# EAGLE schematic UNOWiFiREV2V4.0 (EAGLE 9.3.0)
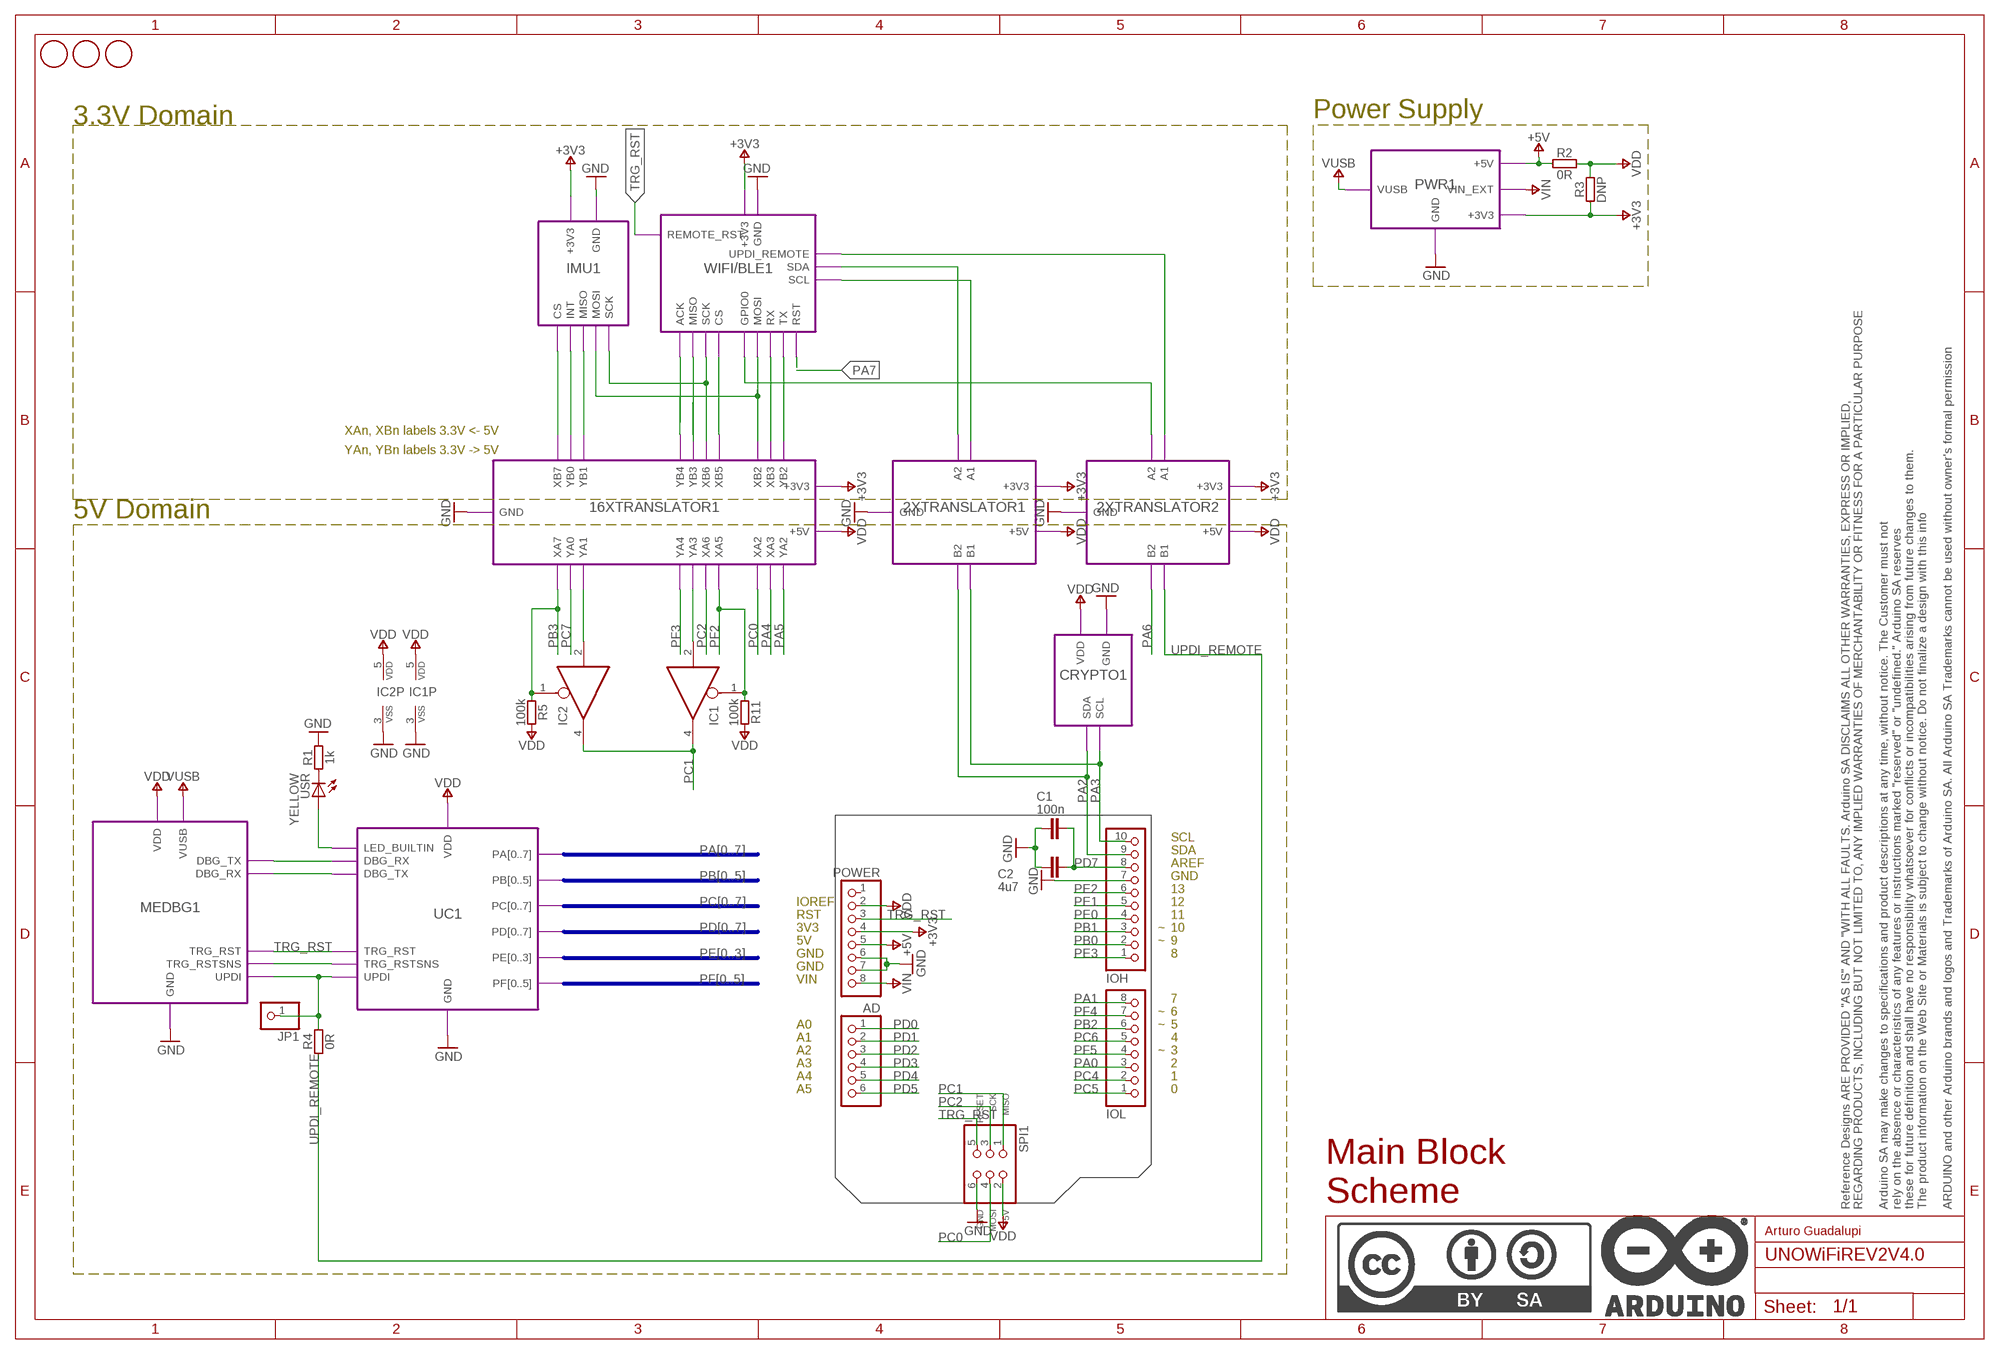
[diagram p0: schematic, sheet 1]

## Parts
AD  Analog  PINHD-1X06TH  [1X06-TH]
C1  100n  C-100NF-0402  [0402-1005X55N]
C2  4u7  C-4.7UF-0402  [0402-1005X55N]
FD1  DNP  FIDUCIAL-2MM  [FD-1-2]
FD2  DNP  FIDUCIAL-2MM  [FD-1-2]
FD3  DNP  FIDUCIAL-2MM  [FD-1-2]
FRAME1  DNP  A3-FRAME  [FRAME]
IC1  74LVC1G125DCKR  SN74LVC1G125DCKR  [SC70-5]
IC2  74LVC1G125DCKR  SN74LVC1G125DCKR  [SC70-5]
IOH  Digital  PINHD-1X10TH  [1X10]
IOL  Digital  PINHD-1X08-DIGITALTH  [1X08]
JP1  PINHD-1X1  [1X01]
POWER  Power  PINHD-1X08-POWERTH  [1X08]
R1  1k  R-1K-0402  [0402-1005X55N]
R2  0R  R-0R-0603  [C0603]
R3  DNP  RDNP-0603  [C0603]
R4  0R  R-0R-0402  [0402-1005X55N]
R5  100k  R-100K-0402  [0402-1005X55N]
R11  100k  R-100K-0402  [0402-1005X55N]
SPI1  -  PINHD-2X03-ICSPTH  [2X03]
USR  YELLOW  LED-YELLOW-0603  [LEDC1608X80N-AK]

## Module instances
UC1 = UC (part numbers offset by 900)
CRYPTO1 = CRYPTO (part numbers offset by 700)
MEDBG1 = MEDBG (part numbers offset by 800)
IMU1 = IMU (part numbers offset by 200)
2XTRANSLATOR1 = 2XTRANSLATOR (part numbers offset by 600)
WIFI/BLE1 = WIFI/BLE (part numbers offset by 300)
PWR1 = PWR (part numbers offset by 100)
16XTRANSLATOR1 = 16XTRANSLATOR (part numbers offset by 500)
2XTRANSLATOR2 = 2XTRANSLATOR (part numbers offset by 400)

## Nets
+3V3: POWER.4 R3.1 ; port WIFI/BLE1.+3V3 2XTRANSLATOR1.+3V3 PWR1.+3V3 IMU1.+3V3 16XTRANSLATOR1.+3V3 2XTRANSLATOR2.+3V3
+5V: POWER.5 R2.1 ; port PWR1.+5V
GND: C1.2 C2.2 IC1.3(VSS) IC2.3(VSS) IOH.7 POWER.6 POWER.7 R1.2 SPI1.6 ; port WIFI/BLE1.GND CRYPTO1.GND PWR1.GND MEDBG1.GND UC1.GND IMU1.GND 16XTRANSLATOR1.GND 2XTRANSLATOR1.GND 2XTRANSLATOR2.GND
N$1: port 2XTRANSLATOR2.A1 WIFI/BLE1.UPDI_REMOTE
N$2: port WIFI/BLE1.MISO 16XTRANSLATOR1.YB3
N$3: port WIFI/BLE1.TX 16XTRANSLATOR1.YB2
N$4: port IMU1.MOSI WIFI/BLE1.MOSI 16XTRANSLATOR1.XB2
N$5: port WIFI/BLE1.RX 16XTRANSLATOR1.XB3
N$6: port IMU1.MISO 16XTRANSLATOR1.YB1
N$7: port WIFI/BLE1.GPIO0 2XTRANSLATOR2.A2
N$8: port WIFI/BLE1.CS 16XTRANSLATOR1.XB5
N$9: IC1.2(I) ; port 16XTRANSLATOR1.YA3 16XTRANSLATOR1.YA3
N$10: IC2.2(I) ; port 16XTRANSLATOR1.YA1
N$12: port WIFI/BLE1.SCL 2XTRANSLATOR1.A1
N$13: port WIFI/BLE1.SDA 2XTRANSLATOR1.A2
N$14: JP1.1 R4.2 ; port UC1.UPDI MEDBG1.UPDI
N$15: port IMU1.INT 16XTRANSLATOR1.YB0
N$16: port IMU1.CS 16XTRANSLATOR1.XB7
N$17: port UC1.TRG_RSTSNS MEDBG1.TRG_RSTSNS
N$18: port WIFI/BLE1.ACK 16XTRANSLATOR1.YB4
N$19: port UC1.DBG_TX MEDBG1.DBG_RX
N$20: port MEDBG1.DBG_TX UC1.DBG_RX
N$21: USR.A ; port UC1.LED_BUILTIN
N$22: R1.1 USR.C
N$23: port IMU1.SCK WIFI/BLE1.SCK 16XTRANSLATOR1.XB6
PA0: IOL.3
PA1: IOL.8
PA2: IOH.9 ; port CRYPTO1.SDA 2XTRANSLATOR1.B2
PA3: IOH.10 ; port CRYPTO1.SCL 2XTRANSLATOR1.B1
PA4: port 16XTRANSLATOR1.XA3
PA5: port 16XTRANSLATOR1.YA2
PA6: port 2XTRANSLATOR2.B2
PA7: port WIFI/BLE1.RST
PB0: IOH.2
PB1: IOH.3
PB2: IOL.6
PB3: IC2.1(OE) R5.1 ; port 16XTRANSLATOR1.XA7
PC0: SPI1.4 ; port 16XTRANSLATOR1.XA2
PC1: IC1.4(O) IC2.4(O) SPI1.1
PC2: SPI1.3 ; port 16XTRANSLATOR1.XA6
PC4: IOL.2
PC5: IOL.1
PC6: IOL.5
PC7: port 16XTRANSLATOR1.YA0
PD0: AD.1
PD1: AD.2
PD2: AD.3
PD3: AD.4
PD4: AD.5
PD5: AD.6
PD7: C1.1 C2.1 IOH.8
PE0: IOH.4
PE1: IOH.5
PE2: IOH.6
PE3: IOH.1
PF2: IC1.1(OE) R11.1 ; port 16XTRANSLATOR1.XA5
PF3: port 16XTRANSLATOR1.YA4
PF4: IOL.7
PF5: IOL.4
TRG_RST: POWER.3 SPI1.5 ; port MEDBG1.TRG_RST UC1.TRG_RST WIFI/BLE1.REMOTE_RST
UPDI_REMOTE: R4.1 ; port 2XTRANSLATOR2.B1
VDD: IC1.5(VDD) IC2.5(VDD) POWER.2 R2.2 R3.2 R5.2 R11.2 SPI1.2 ; port CRYPTO1.VDD MEDBG1.VDD UC1.VDD 16XTRANSLATOR1.+5V 2XTRANSLATOR1.+5V 2XTRANSLATOR2.+5V
VIN: POWER.8 ; port PWR1.VIN_EXT
VUSB: port PWR1.VUSB MEDBG1.VUSB
Unconnected: POWER.1

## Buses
PA[0..7]
PB[0..5]
PC[0..7]
PD[0..7]
PE[0..3]
PF[0..5]

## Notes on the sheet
- 3.3V Domain | Power Supply
- XAn, XBn labels 3.3V <- 5V
- YAn, YBn labels 3.3V -> 5V
- 5V Domain
- SCL
- SDA
- AREF
- GND
- 13
- IOREF | 12
- RST | 11
- 3V3 | ~ | 10
- 5V | ~ | 9
- GND | 8
- GND
- VIN
- 7
- ~ | 6
- A0 | ~ | 5
- A1 | 4
- A2 | ~ | 3
- A3 | 2
- A4 | 1
- A5 | 0
- Main Block 
  Scheme
- Arturo Guadalupi

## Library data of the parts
AD = Arduino-connectors:PINHD-1X06: PIN HEADER; CODE-ARDUINO: 3649; DATASHEET: -; DISTRIBUTOR-LINK: -; DISTRIBUTOR-PN: -; MANUFACTURER: -; MANUFACTURER-PN: FH254-106DF085149V
C1 = Arduino-rcl:C: SMD Capacitor; CODE-ARDUINO: 0132; DATASHEET: http://www.tdk.com/pdf/TDKMLCCCapRange.pdf; DISTRIBUTOR-LINK: http://www.digikey.com/product-detail/en/tdk-corporation/C1005X5R1H104K050BB/445-5942-1-ND/2443982; DISTRIBUTOR-PN: 445-5942-1-ND; MANUFACTURER: TDK; MANUFACTURER-PN: C1005X5R1H104K050BB; NOTE: -
C2 = Arduino-rcl:C: SMD Capacitor; CODE-ARDUINO: 0833; DATASHEET: http://search.murata.co.jp/Ceramy/image/img/A01X/partnumbering_e_01.pdf; DISTRIBUTOR-LINK: http://www.digikey.com/product-detail/en/murata-electronics-north-america/GRM155R60J475ME47D/490-5915-1-ND/3719860; DISTRIBUTOR-PN: 490-5915-1-ND; MANUFACTURER: Murata; MANUFACTURER-PN: GRM155R60J475ME47D; NOTE: -
FD1-FD3 = Arduino-utility:FIDUCIAL: Fiducial mount; CODE-ARDUINO: DNP; DATASHEET: DNP; DISTRIBUTOR-LINK: DNP; DISTRIBUTOR-PN: DNP; MANUFACTURER: DNP; MANUFACTURER-PN: DNP
FRAME1 = Arduino-utility:A3-FRAME; CODE-ARDUINO: DNP; DATASHEET: DNP; DISTRIBUTOR-LINK: DNP; DISTRIBUTOR-PN: DNP; MANUFACTURER: DNP; MANUFACTURER-PN: DNP; NOTE: DNP
IC1 IC2 = Arduino-ICs:SN74LVC1G125DCKR: Single bus buffer with 3-state output; CODE-ARDUINO: 0040; DATASHEET: http://www.ti.com/lit/ds/symlink/sn74lvc1g125.pdf; DISTRIBUTOR-LINK: https://www.digikey.com/product-detail/en/texas-instruments/SN74LVC1G125DCKR/296-11604-1-ND/385743; DISTRIBUTOR-PN: 296-11604-1-ND; MANUFACTURER: Texas Instruments; MANUFACTURER-PN: SN74LVC1G125DCKR; NOTE: NO
IOH = Arduino-connectors:PINHD-1X10: PIN HEADER; CODE-ARDUINO: 3648; DATASHEET: -; DISTRIBUTOR-LINK: -; DISTRIBUTOR-PN: -; MANUFACTURER: -; MANUFACTURER-PN: FH254-110DF085149V
IOL = Arduino-connectors:PINHD-1X08: PIN HEADER; CODE-ARDUINO: 3648; DATASHEET: -; DISTRIBUTOR-LINK: -; DISTRIBUTOR-PN: -; MANUFACTURER: -; MANUFACTURER-PN: FH254-108DF085149V
JP1 = pinhead:PINHD-1X1: PIN HEADER
POWER = Arduino-connectors:PINHD-1X08: PIN HEADER; CODE-ARDUINO: 3649; DATASHEET: -; DISTRIBUTOR-LINK: -; DISTRIBUTOR-PN: -; MANUFACTURER: -; MANUFACTURER-PN: FH254-108DF085149V
R1 = Arduino-rcl:R: SMD Resistor; CODE-ARDUINO: 0140; DATASHEET: www.yageo.com.tw/exep/pages/download/literatures/PYu-R_INT-thick_7.pdf; DISTRIBUTOR-LINK: http://www.digikey.com/product-detail/en/yageo/RC0402FR-071KL/311-1.00KLRCT-ND/729460; DISTRIBUTOR-PN: 311-1.00KLRCT-ND; MANUFACTURER: Yageo; MANUFACTURER-PN: RC0402FR-071KL; NOTE: NO
R2 = Arduino-rcl:R: SMD Resistor; CODE-ARDUINO: 0233; DATASHEET: http://www.yageo.com/exep/pages/download/literatures/PYu-R_Marking_2.pdf; DISTRIBUTOR-LINK: https://www.digikey.com/product-detail/en/yageo/RC0603JR-070RL/311-0.0GRCT-ND/729622; DISTRIBUTOR-PN: 311-0.0GRCT-ND; MANUFACTURER: Yageo; MANUFACTURER-PN: RC0603JR-070RL; NOTE: NO
R3 = Arduino-rcl:R: SMD Resistor; CODE-ARDUINO: DNP; DATASHEET: DNP; DISTRIBUTOR-LINK: DNP; DISTRIBUTOR-PN: DNP; MANUFACTURER: DNP; MANUFACTURER-PN: DNP; NOTE: DNP
R4 = Arduino-rcl:R: SMD Resistor; CODE-ARDUINO: 0039; DATASHEET: www.yageo.com.tw/exep/pages/download/literatures/PYu-R_INT-thick_7.pdf; DISTRIBUTOR-LINK: http://www.digikey.com/product-detail/en/yageo/RC0402FR-070RL/311-0.0LRCT-ND/2827888; DISTRIBUTOR-PN: 311-0.0LRCT-ND; MANUFACTURER: Yageo; MANUFACTURER-PN: RC0402FR-070RL; NOTE: NO
R5 R11 = Arduino-rcl:R: SMD Resistor; CODE-ARDUINO: 0134; DATASHEET: www.yageo.com.tw/exep/pages/download/literatures/PYu-R_INT-thick_7.pdf; DISTRIBUTOR-LINK: http://www.digikey.com/product-detail/en/yageo/RC0402FR-07100KL/311-100KLRCT-ND/729473; DISTRIBUTOR-PN: 311-100KLRCT-ND; MANUFACTURER: Yageo; MANUFACTURER-PN: RC0402FR-07100KL; NOTE: NO
SPI1 = Arduino-connectors:PINHD-2X03-ICSP: PIN HEADER; CODE-ARDUINO: 0114; DATASHEET: -; DISTRIBUTOR-LINK: https://www.digikey.com/product-detail/en/samtec-inc/TSW-103-25-S-D/TSW-103-25-S-D-ND/7863771; DISTRIBUTOR-PN: TSW-103-25-S-D-ND; MANUFACTURER: Samtec; MANUFACTURER-PN: TSW-103-25-S-D
USR = Arduino-diodes:LED: LED; CODE-ARDUINO: 2243; DATASHEET: http://media.digikey.com/pdf/Data%20Sheets/Avago%20PDFs/HSMz-Czzz.pdf; DISTRIBUTOR-LINK: http://www.digikey.com/product-detail/en/broadcom-limited/HSMY-C190/516-1424-1-ND/637748; DISTRIBUTOR-PN: 516-1424-1-ND; MANUFACTURER: Avago; MANUFACTURER-PN: HSMY-C190

## Module UC
Ports: TRG_RSTSNS(out) UPDI(in) TRG_RST(in) GND(pwr) VDD(pwr) DBG_TX(out) DBG_RX(in) LED_BUILTIN(out) PC[0..7](io) PA[0..7](io) PB[0..5](io) PD[0..7](io) PE[0..3](io) PF[0..5](io)
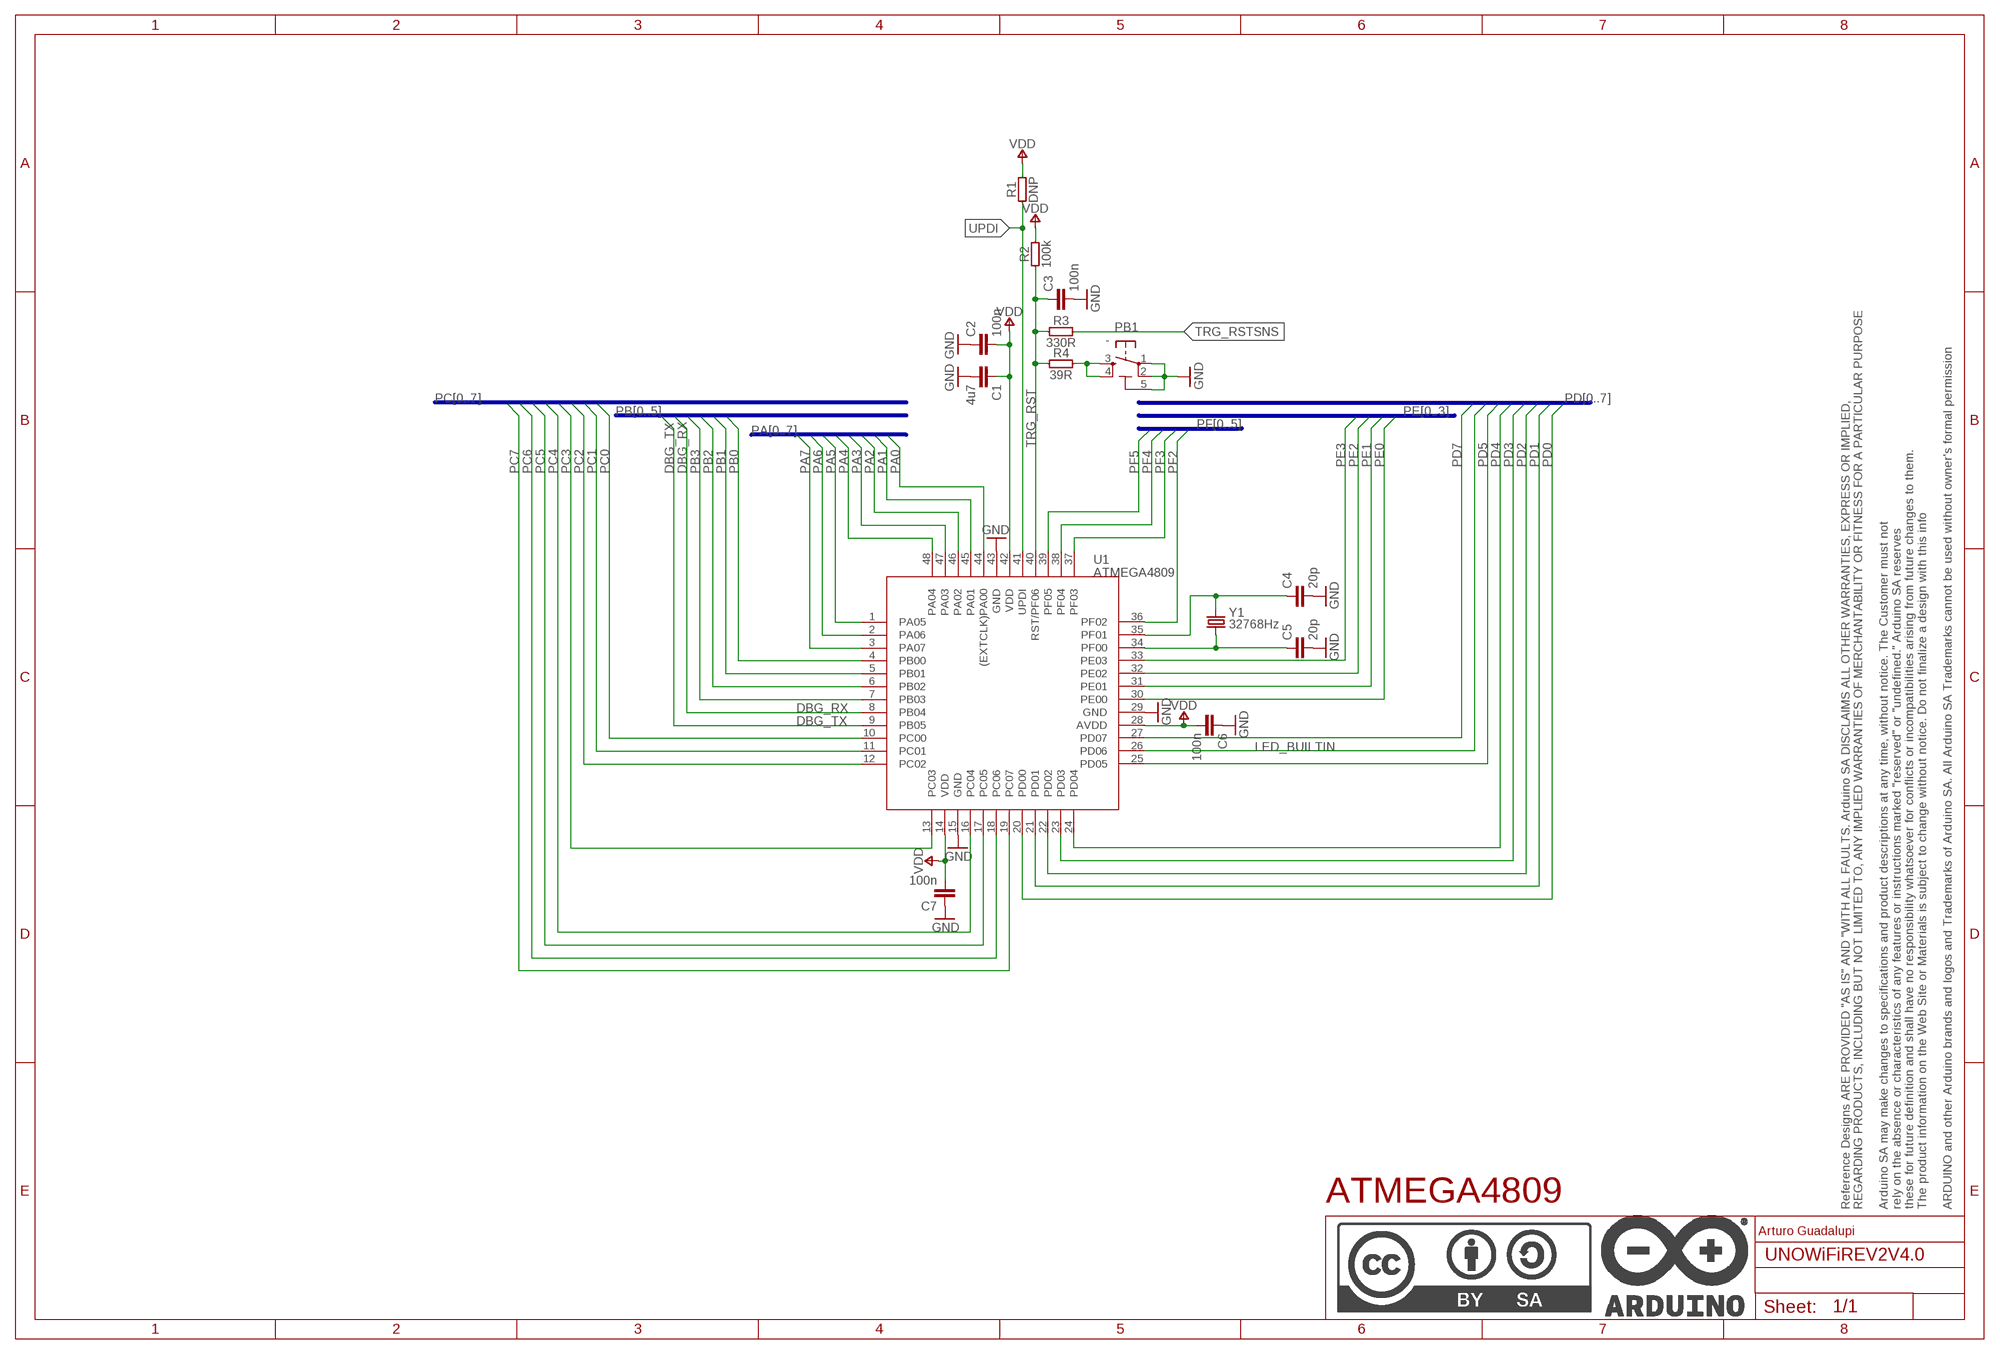
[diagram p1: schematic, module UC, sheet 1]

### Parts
C1  4u7  C-4.7UF-0402  [0402-1005X55N]
C2  100n  C-100NF-0402  [0402-1005X55N]
C3  100n  C-100NF-0402  [0402-1005X55N]
C4  20p  C-20PF-0402  [0402-1005X55N]
C5  20p  C-20PF-0402  [0402-1005X55N]
C6  100n  C-100NF-0402  [0402-1005X55N]
C7  100n  C-100NF-0402  [0402-1005X55N]
FRAME1  DNP  A3-FRAME  [FRAME]
PB1  -  TACTILE2  [TS42]
R1  DNP  R-DNP-0402  [0402-1005X55N]
R2  100k  R-100K-0402  [0402-1005X55N]
R3  330R  R-330R-0402  [0402-1005X55N]
R4  39R  R-39R-0402  [0402-1005X55N]
U1  ATMEGA4809  [TQFP48]
Y1  32768Hz  32.768KHZ  [ABS07]

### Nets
DBG_RX: U1.8(PB04)
DBG_TX: U1.9(PB05)
GND: C1.2 C2.1 C3.2 C4.2 C5.2 C6.1 C7.1 PB1.1 PB1.2 PB1.5(5-GND) U1.15(GND) U1.29(GND) U1.43(GND)
LED_BUILTIN: U1.26(PD06)
N$2: PB1.3 PB1.4 R4.2
N$3: C5.1 U1.34(PF00) Y1.1
N$4: C4.1 U1.35(PF01) Y1.2
PA0: U1.44((EXTCLK)PA00)
PA1: U1.45(PA01)
PA2: U1.46(PA02)
PA3: U1.47(PA03)
PA4: U1.48(PA04)
PA5: U1.1(PA05)
PA6: U1.2(PA06)
PA7: U1.3(PA07)
PB0: U1.4(PB00)
PB1: U1.5(PB01)
PB2: U1.6(PB02)
PB3: U1.7(PB03)
PC0: U1.10(PC00)
PC1: U1.11(PC01)
PC2: U1.12(PC02)
PC3: U1.13(PC03)
PC4: U1.16(PC04)
PC5: U1.17(PC05)
PC6: U1.18(PC06)
PC7: U1.19(PC07)
PD0: U1.20(PD00)
PD1: U1.21(PD01)
PD2: U1.22(PD02)
PD3: U1.23(PD03)
PD4: U1.24(PD04)
PD5: U1.25(PD05)
PD7: U1.27(PD07)
PE0: U1.30(PE00)
PE1: U1.31(PE01)
PE2: U1.32(PE02)
PE3: U1.33(PE03)
PF2: U1.36(PF02)
PF3: U1.37(PF03)
PF4: U1.38(PF04)
PF5: U1.39(PF05)
TRG_RST: C3.1 R2.1 R3.1 R4.1 U1.40(RST/PF06)
TRG_RSTSNS: R3.2
UPDI: R1.1 U1.41(UPDI)
VDD: C1.1 C2.2 C6.2 C7.2 R1.2 R2.2 U1.14(VDD) U1.28(AVDD) U1.42(VDD)

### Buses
PA[0..7]
PB[0..5]
PF[0..5]
PE[0..3]
PD[0..7]
PC[0..7]

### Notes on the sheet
- ATMEGA4809
- Arturo Guadalupi

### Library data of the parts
C1 = Arduino-rcl:C: SMD Capacitor; CODE-ARDUINO: 0833; DATASHEET: http://search.murata.co.jp/Ceramy/image/img/A01X/partnumbering_e_01.pdf; DISTRIBUTOR-LINK: http://www.digikey.com/product-detail/en/murata-electronics-north-america/GRM155R60J475ME47D/490-5915-1-ND/3719860; DISTRIBUTOR-PN: 490-5915-1-ND; MANUFACTURER: Murata; MANUFACTURER-PN: GRM155R60J475ME47D; NOTE: -
C2 C3 C6 C7 = Arduino-rcl:C: SMD Capacitor; CODE-ARDUINO: 0132; DATASHEET: http://www.tdk.com/pdf/TDKMLCCCapRange.pdf; DISTRIBUTOR-LINK: http://www.digikey.com/product-detail/en/tdk-corporation/C1005X5R1H104K050BB/445-5942-1-ND/2443982; DISTRIBUTOR-PN: 445-5942-1-ND; MANUFACTURER: TDK; MANUFACTURER-PN: C1005X5R1H104K050BB; NOTE: -
C4 C5 = Arduino-rcl:C: SMD Capacitor; CODE-ARDUINO: 2188; DATASHEET: http://www.kemet.com/docfinder?Partnumber=CBR04C200J5GAC; DISTRIBUTOR-LINK: http://www.digikey.com/product-detail/en/kemet/CBR04C200J5GAC/399-6173-1-ND/2732143; DISTRIBUTOR-PN: 399-6173-1-ND; MANUFACTURER: Kemet; MANUFACTURER-PN: CBR04C200J5GAC; NOTE: -
FRAME1 = Arduino-utility:A3-FRAME; CODE-ARDUINO: DNP; DATASHEET: DNP; DISTRIBUTOR-LINK: DNP; DISTRIBUTOR-PN: DNP; MANUFACTURER: DNP; MANUFACTURER-PN: DNP; NOTE: DNP
PB1 = Arduino-pushbuttons:TACTILE2: Pushbutton; CODE-ARDUINO: 0946; DATASHEET: http://www.mouser.com/ds/2/418/NG_CD_1571636_C1-122399.pdf; DISTRIBUTOR-LINK: https://www.mouser.it/ProductDetail/TE-Connectivity/1571636-3/?qs=%2fha2pyFaduiys%2fNUBzym%252bcoSb9tuK3Sjuv54qjf0hQ0%3d; DISTRIBUTOR-PN: 506-1571636-3; MANUFACTURER: TE; MANUFACTURER-PN: 1571636-3; PN-ALTERNATIVE1: TS42031-160WWS027260
R1 = Arduino-rcl:R: SMD Resistor; CODE-ARDUINO: DNP; DATASHEET: DNP; DISTRIBUTOR-LINK: DNP; DISTRIBUTOR-PN: DNP; MANUFACTURER: DNP; MANUFACTURER-PN: DNP; NOTE: NO
R2 = Arduino-rcl:R: SMD Resistor; CODE-ARDUINO: 0134; DATASHEET: www.yageo.com.tw/exep/pages/download/literatures/PYu-R_INT-thick_7.pdf; DISTRIBUTOR-LINK: http://www.digikey.com/product-detail/en/yageo/RC0402FR-07100KL/311-100KLRCT-ND/729473; DISTRIBUTOR-PN: 311-100KLRCT-ND; MANUFACTURER: Yageo; MANUFACTURER-PN: RC0402FR-07100KL; NOTE: NO
R3 = Arduino-rcl:R: SMD Resistor; CODE-ARDUINO: 2229; DATASHEET: www.yageo.com.tw/exep/pages/download/literatures/PYu-R_INT-thick_7.pdf; DISTRIBUTOR-LINK: http://www.digikey.com/product-detail/en/yageo/RC0402FR-07330RL/311-330LRCT-ND/729541; DISTRIBUTOR-PN: 311-330LRCT-ND; MANUFACTURER: Yageo; MANUFACTURER-PN: RC0402FR-07330RL; NOTE: NO
R4 = Arduino-rcl:R: SMD Resistor; CODE-ARDUINO: 0138; DATASHEET: www.yageo.com.tw/exep/pages/download/literatures/PYu-R_INT-thick_7.pdf; DISTRIBUTOR-LINK: http://www.digikey.com/product-detail/en/yageo/RC0402FR-0739RL/311-39.0LRCT-ND/729549; DISTRIBUTOR-PN: 311-39.0LRCT-ND; MANUFACTURER: Yageo; MANUFACTURER-PN: RC0402FR-0739RL; NOTE: NO
U1 = Arduino-ucs&SoCs:ATMEGA4809: ATMEGA4809; CODE-ARDUINO: 2322; DATASHEET: http://ww1.microchip.com/downloads/en/DeviceDoc/40002016A.pdf; DISTRIBUTOR-LINK: https://www.digikey.com/product-detail/en/microchip-technology/ATMEGA4809-AFR/ATMEGA4809-AFRCT-ND/8540756; DISTRIBUTOR-PN: ATMEGA4809-AFRCT-ND; MANUFACTURER: Microchip; MANUFACTURER-PN: ATMEGA4809-AFR
Y1 = Arduino-crystals:32.768KHZ: LF crystal; CODE-ARDUINO: 0213; DATASHEET: http://www.abracon.com/Resonators/ABS07.pdf; DISTRIBUTOR-LINK: http://www.digikey.com/product-detail/en/abracon-llc/ABS07-32.768KHZ-T/535-9542-1-ND/1237009; DISTRIBUTOR-PN: 535-9542-1-ND; MANUFACTURER: Abracon LLC; MANUFACTURER-PN: ABS07-32.768KHZ-T

## Module CRYPTO
Ports: SDA(io) SCL(in) GND(pwr) VDD(pwr)
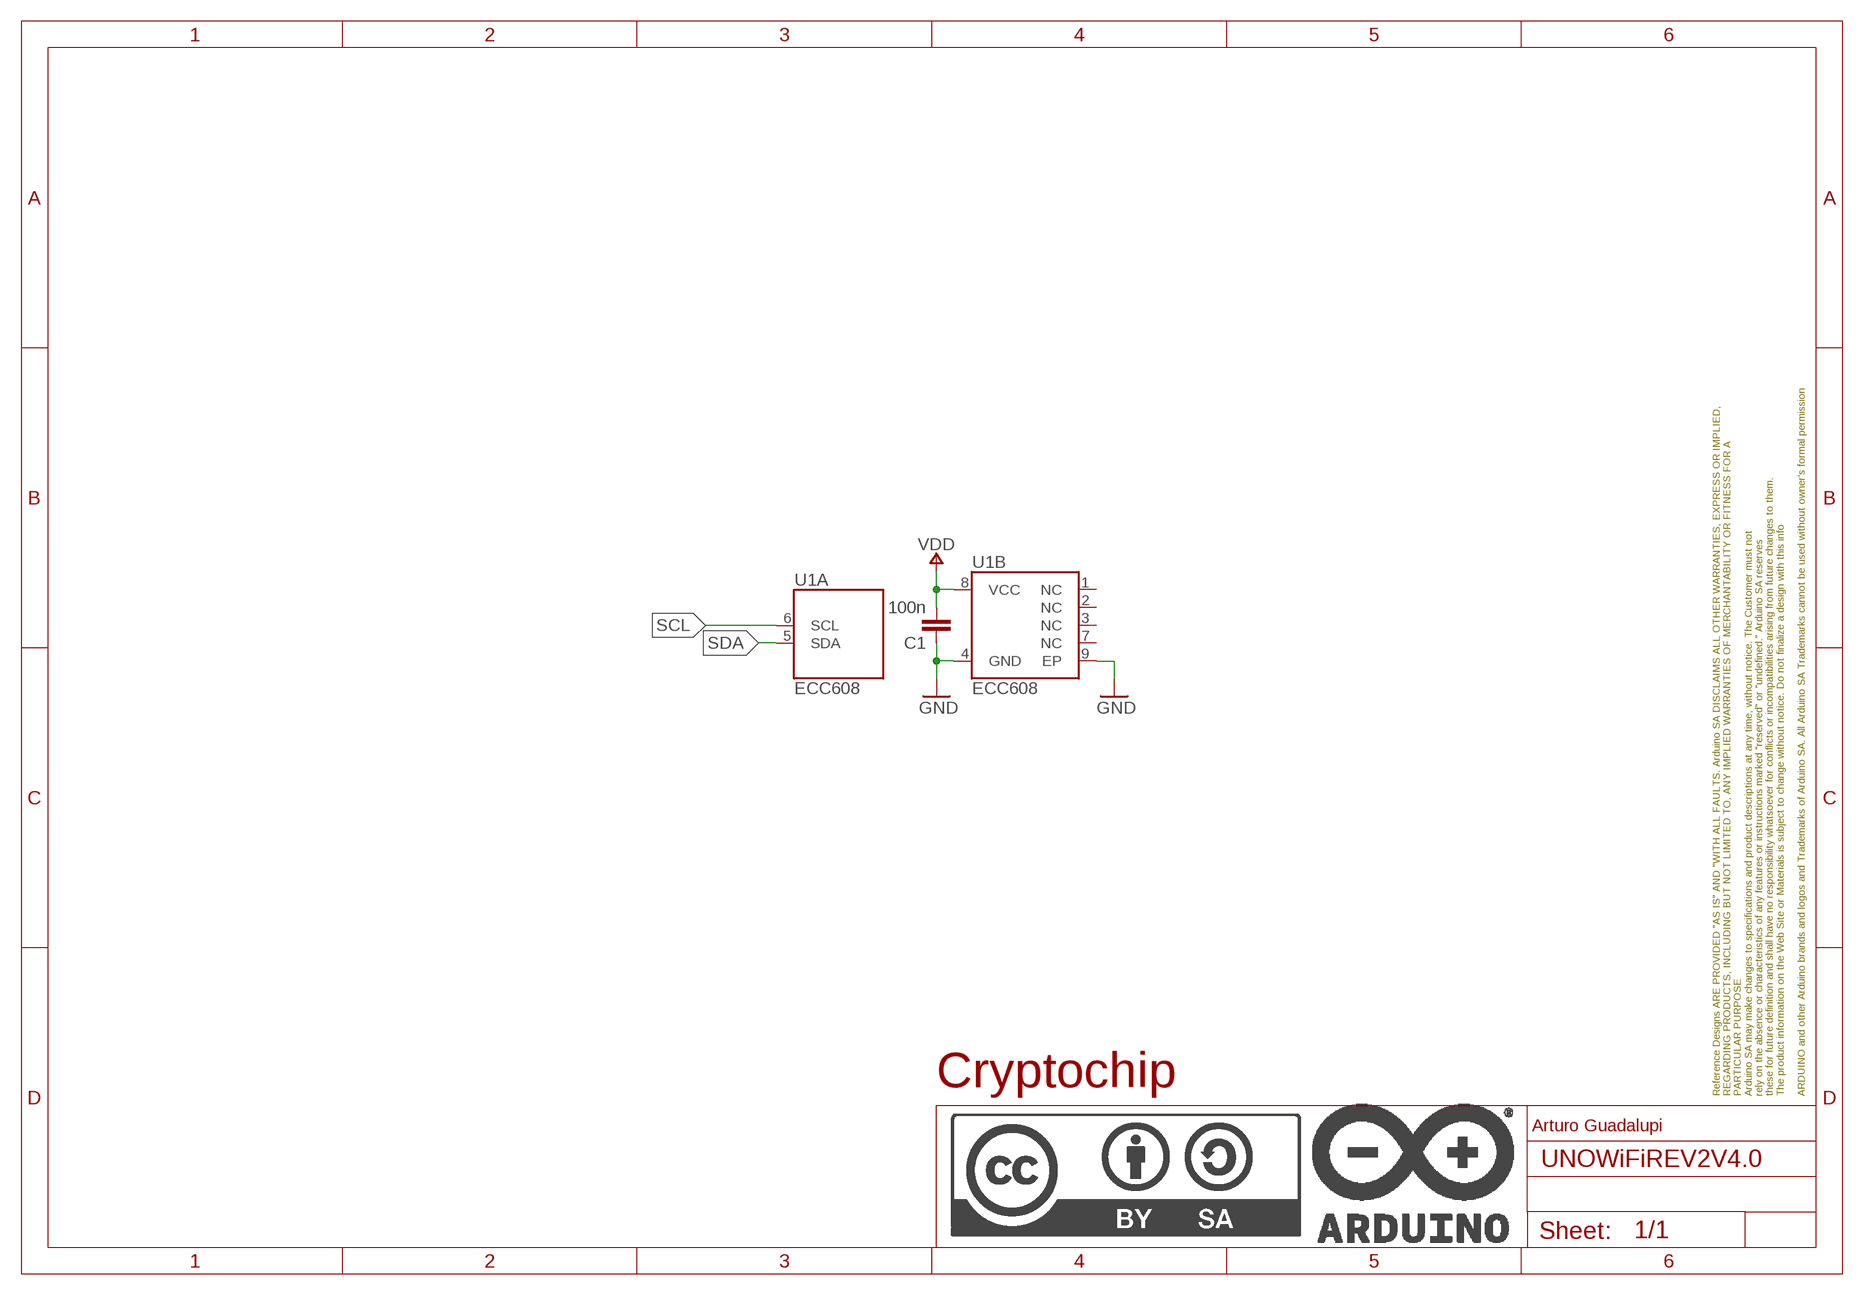
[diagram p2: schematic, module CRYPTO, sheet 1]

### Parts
C1  100n  C-100NF-0402  [0402-1005X55N]
FRAME1  DNP  A4L-LOC  [FRAME]
U1  ECC608  ATECC-6088-UDFN  [SON50P300X200X60-9N-EP160X140]

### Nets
GND: C1.1 U1.4(B:GND) U1.9(B:EP)
SCL: U1.6(A:SCL)
SDA: U1.5(A:SDA)
VDD: C1.2 U1.8(B:VCC)
Unconnected: U1.1(B:NC) U1.2(B:NC) U1.3(B:NC) U1.7(B:NC)

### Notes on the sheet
- Cryptochip
- Arturo Guadalupi

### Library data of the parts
C1 = Arduino-rcl:C: SMD Capacitor; CODE-ARDUINO: 0132; DATASHEET: http://www.tdk.com/pdf/TDKMLCCCapRange.pdf; DISTRIBUTOR-LINK: http://www.digikey.com/product-detail/en/tdk-corporation/C1005X5R1H104K050BB/445-5942-1-ND/2443982; DISTRIBUTOR-PN: 445-5942-1-ND; MANUFACTURER: TDK; MANUFACTURER-PN: C1005X5R1H104K050BB; NOTE: -
FRAME1 = Arduino-utility:A4L-LOC; CODE-ARDUINO: DNP; DATASHEET: DNP; DISTRIBUTOR-LINK: DNP; DISTRIBUTOR-PN: DNP; MANUFACTURER: DNP; MANUFACTURER-PN: DNP; NOTE: DNP
U1 = Arduino-ICs:ATECC: Secure authentication and product validation device, EEPROM, I2C, 2.0 - 5.5V; CODE-ARDUINO: A5007; DATASHEET: http://ww1.microchip.com/downloads/en/DeviceDoc/40001977A.pdf; DISTRIBUTOR-LINK: https://www.digikey.com/product-detail/en/microchip-technology/ATECC608A-MAHDA-T/ATECC608A-MAHDA-TCT-ND/7928236; DISTRIBUTOR-PN: ATECC608A-MAHDA-TCT-ND; MANUFACTURER: Microchip; MANUFACTURER-PN: ATECC608A-MAHDA-T; NOTE: NO

## Module MEDBG
Ports: VDD(pwr) VUSB(pwr) GND(pwr) DBG_TX(out) DBG_RX(in) TRG_RSTSNS(in) TRG_RST(out) UPDI(out)
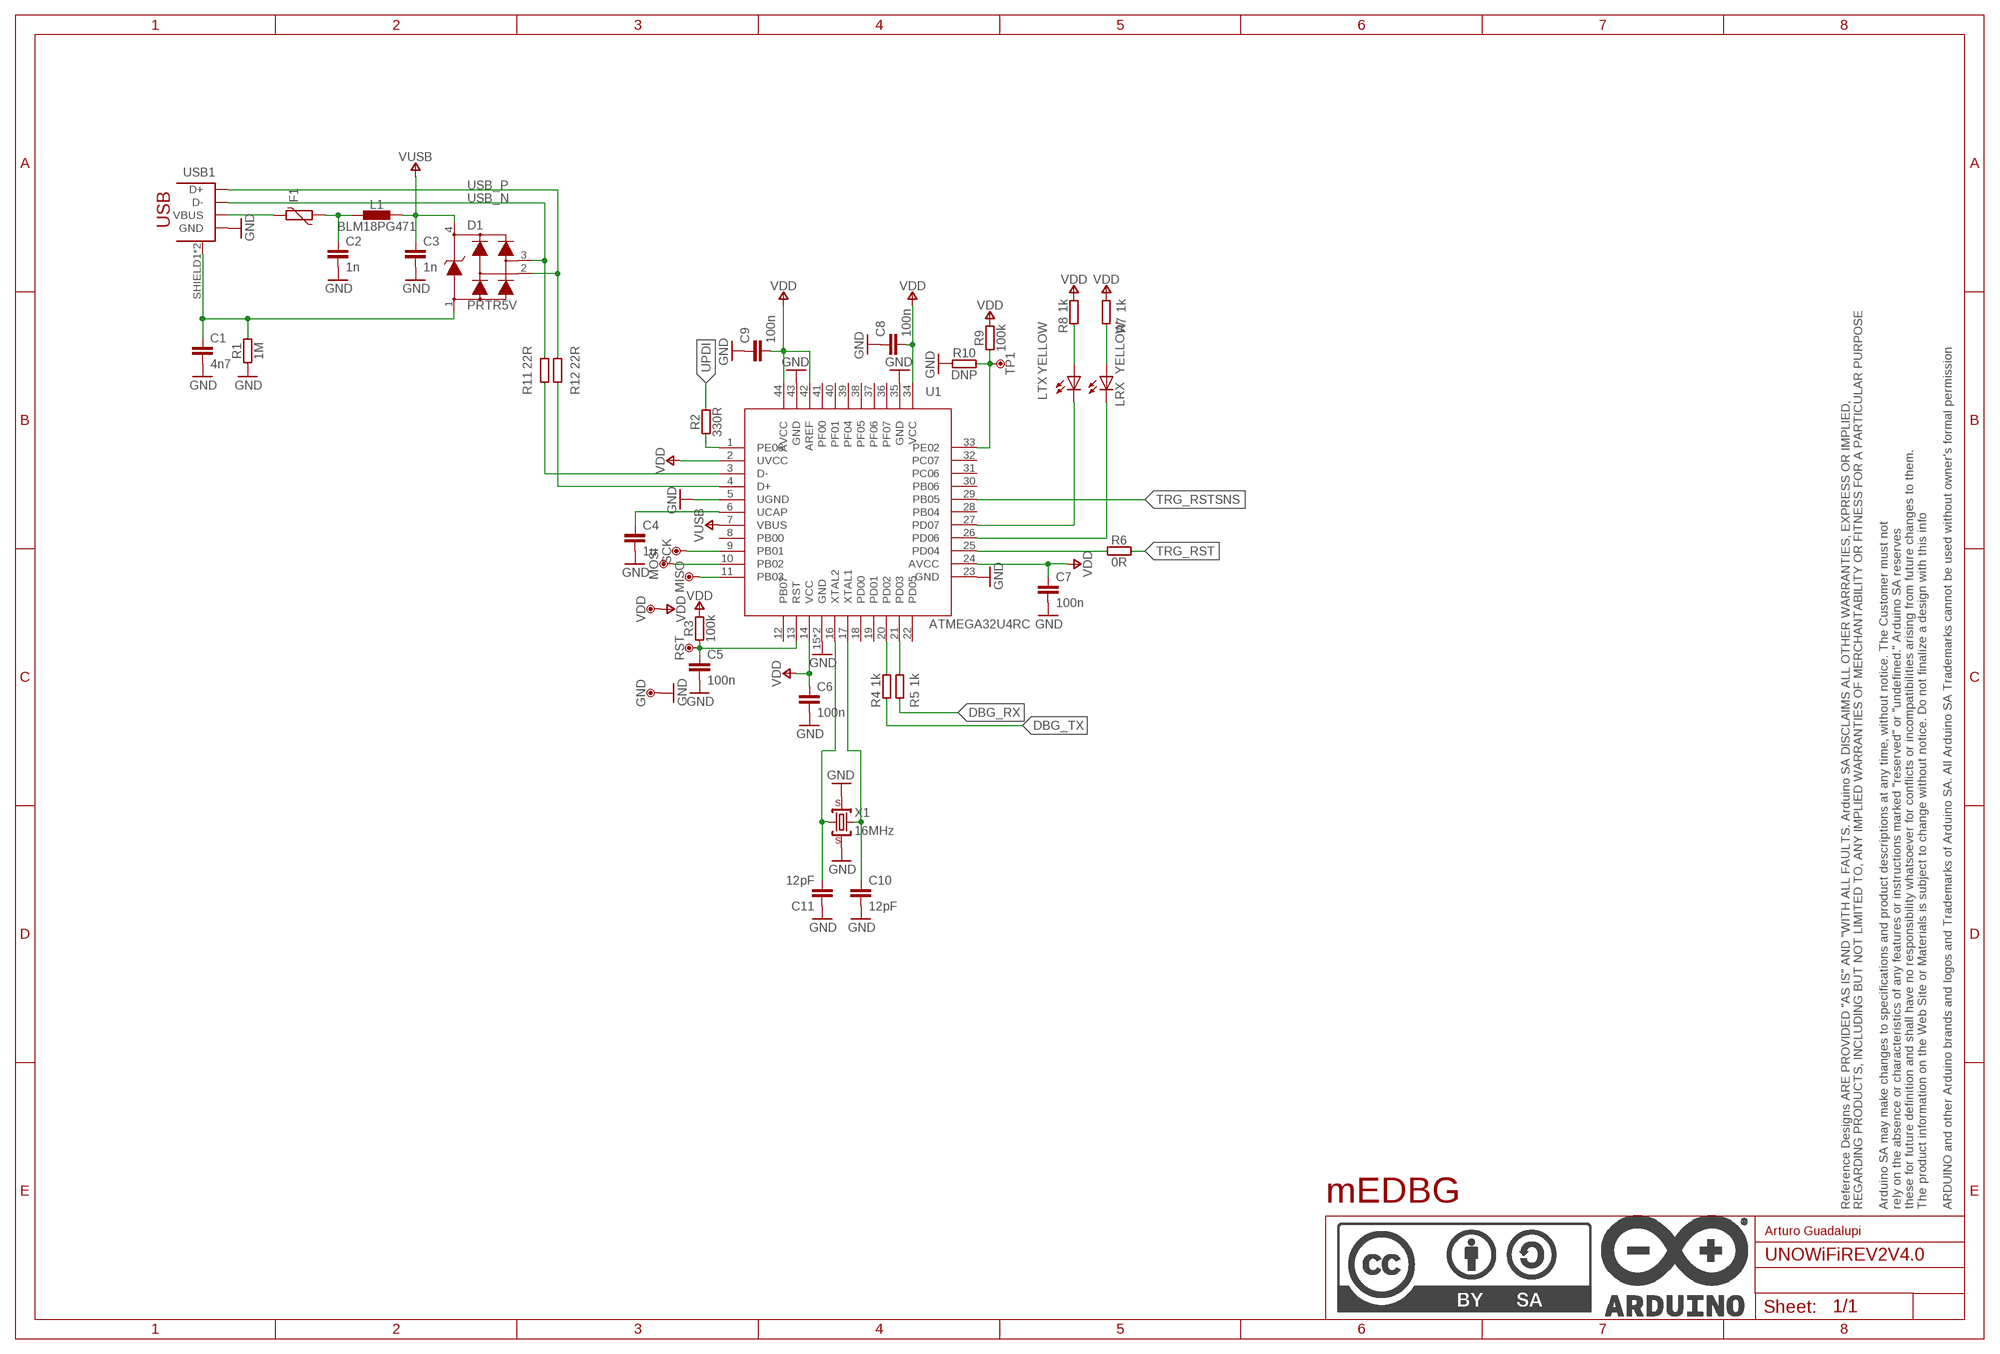
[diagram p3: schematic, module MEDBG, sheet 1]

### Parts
C1  4n7  C4.7NF-0805  [0805-R2013X50N]
C2  1n  C-1NF-0402  [0402-1005X55N]
C3  1n  C-1NF-0402  [0402-1005X55N]
C4  1u  C-1UF-0402  [0402-1005X55N]
C5  100n  C-100NF-0402  [0402-1005X55N]
C6  100n  C-100NF-0402  [0402-1005X55N]
C7  100n  C-100NF-0402  [0402-1005X55N]
C8  100n  C-100NF-0402  [0402-1005X55N]
C9  100n  C-100NF-0402  [0402-1005X55N]
C10  12pF  C-12PF-0402  [0402-1005X55N]
C11  12pF  C-12PF-0402  [0402-1005X55N]
D1  PRTR5V  PRTR5V0U2X,215  [SOT190P230X110-4N]
F1  PTC-0805  [C0805]
FRAME1  DNP  A3-FRAME  [FRAME]
GND  DNP  TPTP-1.00MM  [TP-1.00MM]
L1  BLM18PG471  FERRITE-470R0603  [0603-1608X90N]
LRX  YELLOW  LED-YELLOW-0603  [LEDC1608X80N-AK]
LTX  YELLOW  LED-YELLOW-0603  [LEDC1608X80N-AK]
MISO  DNP  TPTP-1.00MM  [TP-1.00MM]
MOSI  DNP  TPTP-1.00MM  [TP-1.00MM]
R1  1M  R-1M-0402  [0402-1005X55N]
R2  330R  R-330R-0402  [0402-1005X55N]
R3  100k  R-100K-0402  [0402-1005X55N]
R4  1k  R-1K-0402  [0402-1005X55N]
R5  1k  R-1K-0402  [0402-1005X55N]
R6  0R  R-0R-0402  [0402-1005X55N]
R7  1k  R-1K-0402  [0402-1005X55N]
R8  1k  R-1K-0402  [0402-1005X55N]
R9  100k  R-100K-0402  [0402-1005X55N]
R10  DNP  R-DNP-0402  [0402-1005X55N]
R11  22R  R-22R-0402  [0402-1005X55N]
R12  22R  R-22R-0402  [0402-1005X55N]
RST  DNP  TPTP-1.00MM  [TP-1.00MM]
SCK  DNP  TPTP-1.00MM  [TP-1.00MM]
TP1  DNP  TPTP-1.27MM  [TP-1.27MM]
U1  ATMEGA32U4RC  ATMEGA32U4  [QFN50P700X700X100-45N]
USB1  -  USB-B-H  [USB-B-H]
VDD  DNP  TPTP-1.00MM  [TP-1.00MM]
X1  16MHz  CRYSTAL-3.2X2.5-16MHZ(12PF)  [CRYSTAL-3.2-2.5]

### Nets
DBG_RX: R5.1
DBG_TX: R4.1
GND: C1.2 C2.2 C3.2 C4.2 C5.2 C6.2 C7.2 C8.1 C9.1 C10.2 C11.1 GND.X R1.1 R10.1 U1.5(UGND) U1.15(GND) U1.23(GND) U1.35(GND) U1.43(GND) U1.45(GND) USB1.GND X1.2(GND) X1.4(GND)
N$1: C1.1 D1.1 R1.2 USB1.SHIELD1(SHIELD) USB1.SHIELD2(SHIELD)
N$2: F1.2 USB1.VBUS
N$3: C2.1 F1.1 L1.1
N$4: R2.1 U1.1(PE06)
N$5: C4.1 U1.6(UCAP)
N$6: C5.1 R3.1 RST.X U1.13(RST)
N$7: C11.2 U1.16(XTAL2) X1.1(C1)
N$8: C10.1 U1.17(XTAL1) X1.3(C2)
N$9: R4.2 U1.20(PD02)
N$10: R5.2 U1.21(PD03)
N$11: LTX.C U1.27(PD07)
N$12: R6.1 U1.25(PD04)
N$13: LRX.C U1.26(PD06)
N$14: LTX.A R8.1
N$15: LRX.A R7.1
N$16: R9.1 R10.2 TP1.X U1.33(PE02)
N$17: MISO.X U1.11(PB03)
N$18: MOSI.X U1.10(PB02)
N$19: SCK.X U1.9(PB01)
TRG_RST: R6.2
TRG_RSTSNS: U1.29(PB05)
UPDI: R2.2
USB2_N: R11.1 U1.3(D-)
USB2_PI: R12.1 U1.4(D+)
USB_N: D1.3 R11.2 USB1.D-
USB_P: D1.2 R12.2 USB1.D+
VDD: C6.1 C7.1 C8.2 C9.2 R3.2 R7.2 R8.2 R9.2 U1.2(UVCC) U1.14(VCC) U1.24(AVCC) U1.34(VCC) U1.42(AREF) U1.44(AVCC) VDD.X
VUSB: C3.1 D1.4 L1.2 U1.7(VBUS)
Unconnected: U1.8(PB00) U1.12(PB07) U1.18(PD00) U1.19(PD01) U1.22(PD05) U1.28(PB04) U1.30(PB06) U1.31(PC06) U1.32(PC07) U1.36(PF07) U1.37(PF06) U1.38(PF05) U1.39(PF04) U1.40(PF01) U1.41(PF00)

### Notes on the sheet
- mEDBG
- Arturo Guadalupi

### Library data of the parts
C1 = Arduino-rcl:C: SMD Capacitor; CODE-ARDUINO: 0689; DATASHEET: http://www.kemet.com/Lists/ProductCatalog/Attachments/40/KEM_C1010_X7R_HV_SMD.pdf; DISTRIBUTOR-LINK: www.kemet.com/docfinder?Partnumber=C0805C472KDRACTU; DISTRIBUTOR-PN: 399-6738-1-ND; MANUFACTURER: Kemet; MANUFACTURER-PN: C0805C472KDRACTU; NOTE: -
C2 C3 = Arduino-rcl:C: SMD Capacitor; CODE-ARDUINO: 2321; DATASHEET: http://www.samsungsem.com/kr/support/product-search/mlcc/__icsFiles/afieldfile/2016/08/18/S_CL05B102KB5NNNC.pdf; DISTRIBUTOR-LINK: http://www.digikey.com/product-detail/en/samsung-electro-mechanics-america-inc/CL05B102KB5NNNC/1276-1032-1-ND/3889118; DISTRIBUTOR-PN: 1276-1032-1-ND; MANUFACTURER: Samsung; MANUFACTURER-PN: CL05B102KB5NNNC; NOTE: -
C4 = Arduino-rcl:C: SMD Capacitor; CODE-ARDUINO: 0133; DATASHEET: http://search.murata.co.jp/Ceramy/image/img/A01X/partnumbering_e_01.pdf; DISTRIBUTOR-LINK: http://www.digikey.com/product-detail/en/murata-electronics-north-america/GRM155R61E105KA12D/490-10017-1-ND/5026367; DISTRIBUTOR-PN: 490-10017-1-ND; MANUFACTURER: Murata; MANUFACTURER-PN: GRM155R61E105KA12D; NOTE: -
C5-C9 = Arduino-rcl:C: SMD Capacitor; CODE-ARDUINO: 0132; DATASHEET: http://www.tdk.com/pdf/TDKMLCCCapRange.pdf; DISTRIBUTOR-LINK: http://www.digikey.com/product-detail/en/tdk-corporation/C1005X5R1H104K050BB/445-5942-1-ND/2443982; DISTRIBUTOR-PN: 445-5942-1-ND; MANUFACTURER: TDK; MANUFACTURER-PN: C1005X5R1H104K050BB; NOTE: -
C10 C11 = Arduino-rcl:C: SMD Capacitor; CODE-ARDUINO: A5006; DATASHEET: http://search.murata.co.jp/Ceramy/image/img/A01X/partnumbering_e_01.pdf; DISTRIBUTOR-LINK: https://www.digikey.com/product-detail/en/murata-electronics-north-america/GJM1555C1H120GB01D/490-8078-1-ND/4380364; DISTRIBUTOR-PN: 490-8078-1-ND; MANUFACTURER: Murata; MANUFACTURER-PN: GJM1555C1H120GB01D; NOTE: -
D1 = Arduino-diodes:PRTR5V0U2X,215: USB ESD protection; CODE-ARDUINO: 2209; DATASHEET: http://www.nxp.com/documents/data_sheet/PRTR5V0U2X.pdf; DISTRIBUTOR-LINK: http://www.digikey.com/product-detail/en/nxp-semiconductors/PRTR5V0U2X,215/568-4140-1-ND/1589981; DISTRIBUTOR-PN: 568-4140-1-ND; MANUFACTURER: NXP; MANUFACTURER-PN: PRTR5V0U2X,215
F1 = Arduino-rcl:PTC: SMD PTC; CODE-ARDUINO: 0002; DATASHEET: https://www.bourns.com/docs/Product-Datasheets/mfmsmf.pdf; DISTRIBUTOR-LINK: https://www.digikey.it/product-detail/en/bourns-inc/MF-MSMF050-2/MF-MSMF050-2CT-ND/662842; DISTRIBUTOR-PN: MF-MSMF050-2CT-ND; MANUFACTURER: Bourns; MANUFACTURER-PN: MF-MSMF050-2
FRAME1 = Arduino-utility:A3-FRAME; CODE-ARDUINO: DNP; DATASHEET: DNP; DISTRIBUTOR-LINK: DNP; DISTRIBUTOR-PN: DNP; MANUFACTURER: DNP; MANUFACTURER-PN: DNP; NOTE: DNP
GND MISO MOSI RST SCK TP1 VDD = Arduino-utility:TP: Testpoint; CODE-ARDUINO: DNP; DATASHEET: DNP; DISTRIBUTOR-LINK: DNP; DISTRIBUTOR-PN: DNP; MANUFACTURER: DNP; MANUFACTURER-PN: DNP
L1 = Arduino-rcl:FERRITE: SMD ferrite; CODE-ARDUINO: 2217; DATASHEET: http://search.murata.co.jp/Ceramy/image/img/PDF/ENG/L0110S0100BLM18P.pdf; DISTRIBUTOR-LINK: http://www.digikey.com/product-detail/en/murata-electronics-north-america/BLM18PG471SN1D/490-5223-1-ND/1948399; DISTRIBUTOR-PN: 490-5223-1-ND; MANUFACTURER: Murata; MANUFACTURER-PN: BLM18PG471SN1D; NOTE: -
LRX LTX = Arduino-diodes:LED: LED; CODE-ARDUINO: 2243; DATASHEET: http://media.digikey.com/pdf/Data%20Sheets/Avago%20PDFs/HSMz-Czzz.pdf; DISTRIBUTOR-LINK: http://www.digikey.com/product-detail/en/broadcom-limited/HSMY-C190/516-1424-1-ND/637748; DISTRIBUTOR-PN: 516-1424-1-ND; MANUFACTURER: Avago; MANUFACTURER-PN: HSMY-C190
R1 = Arduino-rcl:R: SMD Resistor; CODE-ARDUINO: 0139; DATASHEET: www.yageo.com.tw/exep/pages/download/literatures/PYu-R_INT-thick_7.pdf; DISTRIBUTOR-LINK: http://www.digikey.com/product-detail/en/yageo/RC0402JR-07330RL/311-330JRCT-ND/729412; DISTRIBUTOR-PN: 311-330JRCT-ND; MANUFACTURER: Yageo; MANUFACTURER-PN: RC0402JR-07330RL; NOTE: NO
R2 = Arduino-rcl:R: SMD Resistor; CODE-ARDUINO: 2229; DATASHEET: www.yageo.com.tw/exep/pages/download/literatures/PYu-R_INT-thick_7.pdf; DISTRIBUTOR-LINK: http://www.digikey.com/product-detail/en/yageo/RC0402FR-07330RL/311-330LRCT-ND/729541; DISTRIBUTOR-PN: 311-330LRCT-ND; MANUFACTURER: Yageo; MANUFACTURER-PN: RC0402FR-07330RL; NOTE: NO
R3 R9 = Arduino-rcl:R: SMD Resistor; CODE-ARDUINO: 0134; DATASHEET: www.yageo.com.tw/exep/pages/download/literatures/PYu-R_INT-thick_7.pdf; DISTRIBUTOR-LINK: http://www.digikey.com/product-detail/en/yageo/RC0402FR-07100KL/311-100KLRCT-ND/729473; DISTRIBUTOR-PN: 311-100KLRCT-ND; MANUFACTURER: Yageo; MANUFACTURER-PN: RC0402FR-07100KL; NOTE: NO
R4 R5 R7 R8 = Arduino-rcl:R: SMD Resistor; CODE-ARDUINO: 0140; DATASHEET: www.yageo.com.tw/exep/pages/download/literatures/PYu-R_INT-thick_7.pdf; DISTRIBUTOR-LINK: http://www.digikey.com/product-detail/en/yageo/RC0402FR-071KL/311-1.00KLRCT-ND/729460; DISTRIBUTOR-PN: 311-1.00KLRCT-ND; MANUFACTURER: Yageo; MANUFACTURER-PN: RC0402FR-071KL; NOTE: NO
R6 = Arduino-rcl:R: SMD Resistor; CODE-ARDUINO: 0039; DATASHEET: www.yageo.com.tw/exep/pages/download/literatures/PYu-R_INT-thick_7.pdf; DISTRIBUTOR-LINK: http://www.digikey.com/product-detail/en/yageo/RC0402FR-070RL/311-0.0LRCT-ND/2827888; DISTRIBUTOR-PN: 311-0.0LRCT-ND; MANUFACTURER: Yageo; MANUFACTURER-PN: RC0402FR-070RL; NOTE: NO
R10 = Arduino-rcl:R: SMD Resistor; CODE-ARDUINO: DNP; DATASHEET: DNP; DISTRIBUTOR-LINK: DNP; DISTRIBUTOR-PN: DNP; MANUFACTURER: DNP; MANUFACTURER-PN: DNP; NOTE: NO
R11 R12 = Arduino-rcl:R: SMD Resistor; CODE-ARDUINO: 0468; DATASHEET: www.yageo.com.tw/exep/pages/download/literatures/PYu-R_INT-thick_7.pdf; DISTRIBUTOR-LINK: http://www.digikey.com/products/en?keywords=311-22.0LRCT-ND; DISTRIBUTOR-PN: 311-22.0LRCT-ND; MANUFACTURER: Yageo; MANUFACTURER-PN: RC0402FR-0722RL; NOTE: NO
U1 = Arduino-ucs&SoCs:ATMEGA32U4: ATMEGA32U4; CODE-ARDUINO: 0159; DATASHEET: http://ww1.microchip.com/downloads/en/DeviceDoc/Atmel-7766-8-bit-AVR-ATmega16U4-32U4_Datasheet.pdf; DISTRIBUTOR-LINK: https://www.digikey.com/product-detail/en/microchip-technology/ATMEGA32U4RC-MU/ATMEGA32U4RC-MU-ND/2507984; DISTRIBUTOR-PN: ATMEGA32U4RC-MU-ND; MANUFACTURER: Microchip; MANUFACTURER-PN: ATMEGA32U4RC-MU
USB1 = Arduino-connectors:USB: USB Connectors; CODE-ARDUINO: 0056; DATASHEET: http://cnctech.us/pdfs/1001-003-02000.pdf; DISTRIBUTOR-LINK: https://www.digikey.com/products/it?keywords=1001-003-02000; DISTRIBUTOR-PN: 1175-1002-ND; MANUFACTURER: CNC Tech; MANUFACTURER-PN: 1001-003-02000; PN-ALTERNATIVE1: USB-B-S-RA-WT-SPCC
X1 = Arduino-crystals:CRYSTAL-3.2X2.5: Crystal SMD 3.2x2.5mm; CODE-ARDUINO: 0395; DATASHEET: https://www.ecsxtal.com/store/pdf/ECX-33Q.pdf; DISTRIBUTOR-LINK: https://www.digikey.com/product-detail/en/ecs-inc/ECS-160-12-33Q-JES-TR/XC2147CT-ND/6050976; DISTRIBUTOR-PN: XC2147CT-ND; MANUFACTURER: ECS; MANUFACTURER-PN: ECS-160-12-33Q-JES-TR

## Module IMU
Ports: MOSI(in) SCK(in) MISO(out) INT(out) CS(in) +3V3(pwr) GND(pwr)
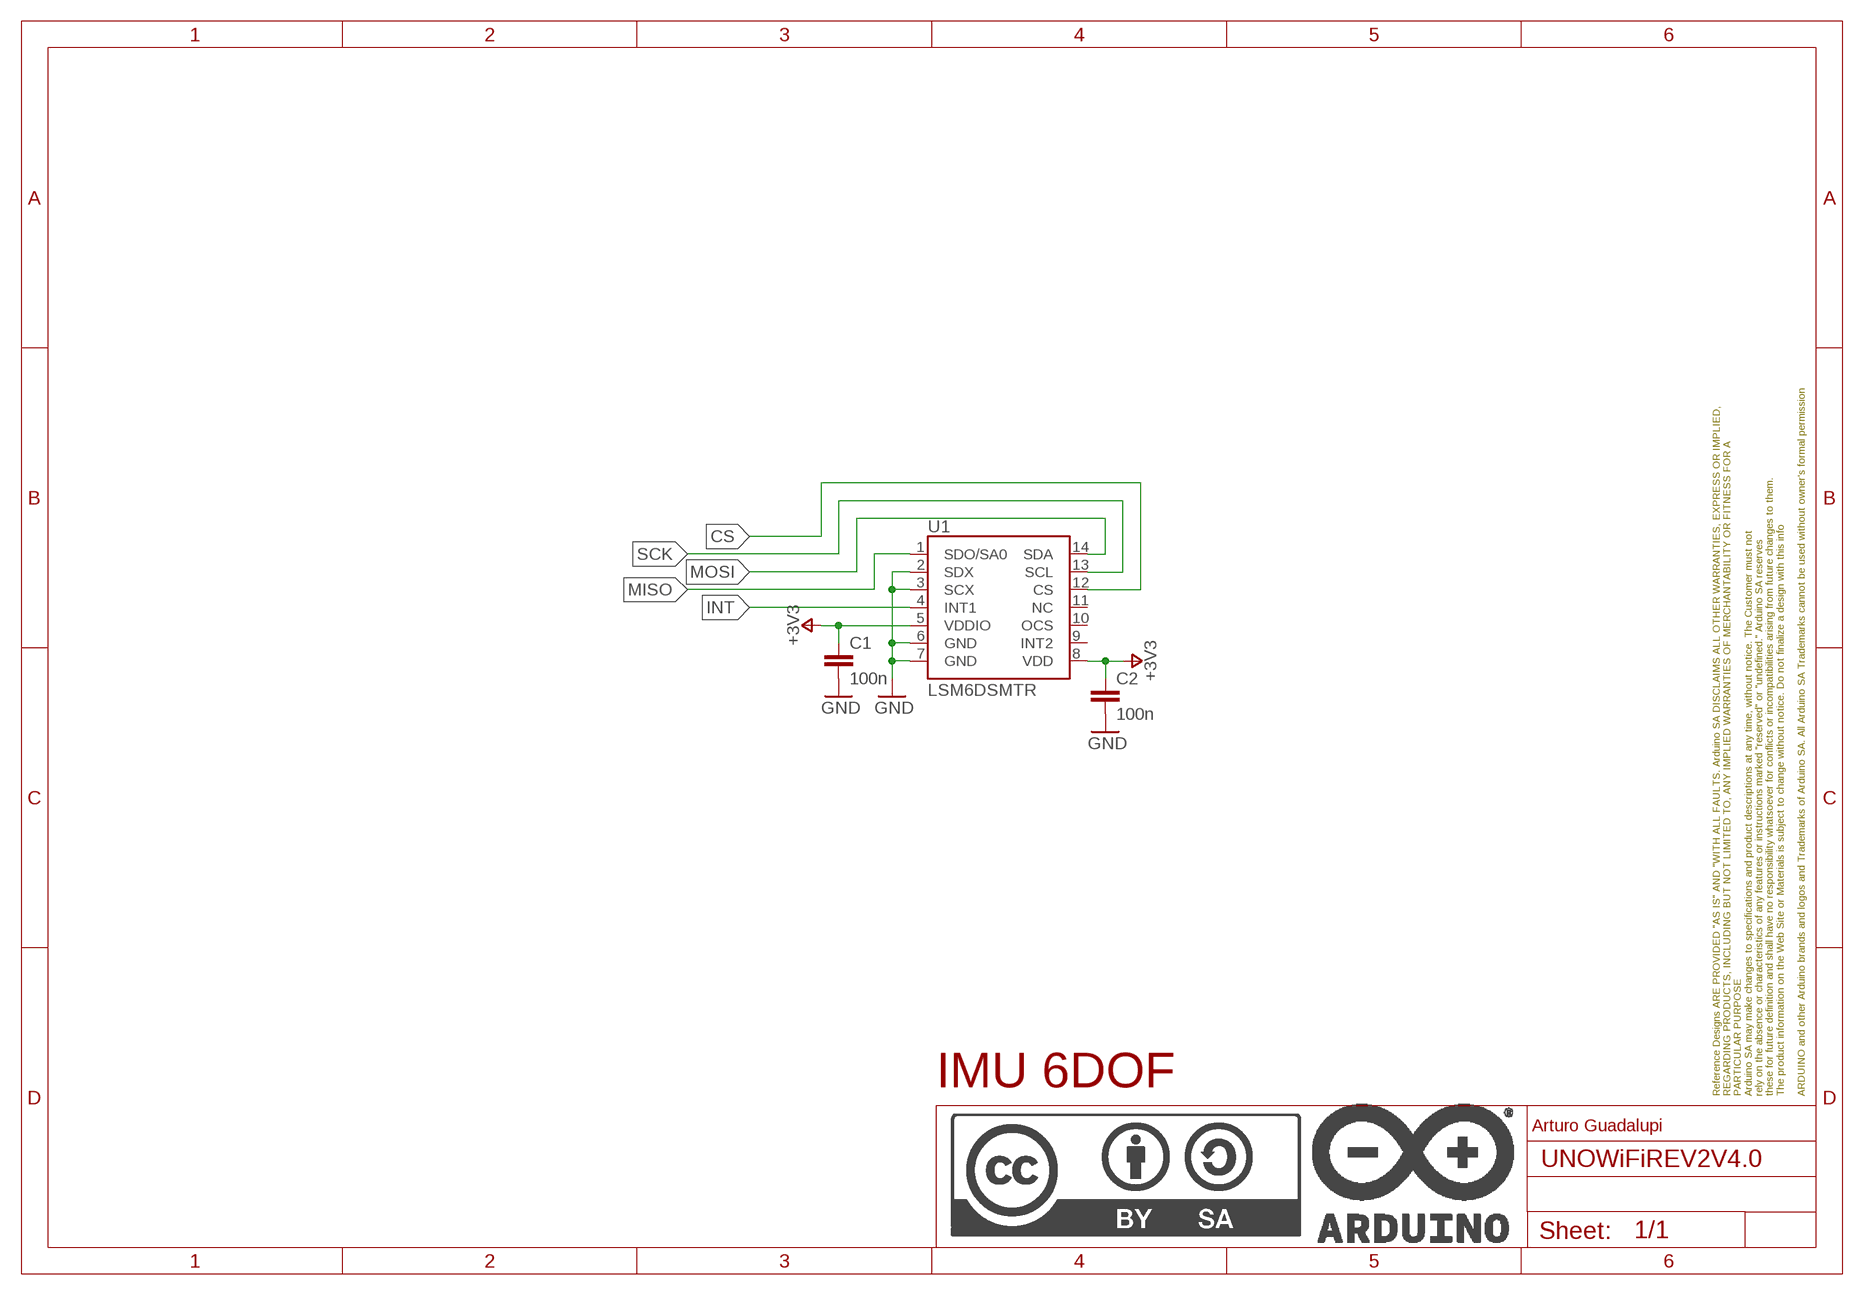
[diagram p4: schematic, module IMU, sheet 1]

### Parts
C1  100n  C-100NF-0402  [0402-1005X55N]
C2  100n  C-100NF-0402  [0402-1005X55N]
FRAME1  DNP  A4L-LOC  [FRAME]
U1  LSM6DSMTR  LSM6DS3LGA  [LGA14L]

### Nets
+3V3: C1.1 C2.1 U1.5(VDDIO) U1.8(VDD)
CS: U1.12(CS)
GND: C1.2 C2.2 U1.2(SDX) U1.3(SCX) U1.6(GND) U1.7(GND)
INT: U1.4(INT1)
MISO: U1.1(SDO/SA0)
MOSI: U1.14(SDA)
SCK: U1.13(SCL)
Unconnected: U1.9(INT2) U1.10(OCS) U1.11(NC)

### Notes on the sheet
- IMU 6DOF
- Arturo Guadalupi

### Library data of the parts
C1 C2 = Arduino-rcl:C: SMD Capacitor; CODE-ARDUINO: 0132; DATASHEET: http://www.tdk.com/pdf/TDKMLCCCapRange.pdf; DISTRIBUTOR-LINK: http://www.digikey.com/product-detail/en/tdk-corporation/C1005X5R1H104K050BB/445-5942-1-ND/2443982; DISTRIBUTOR-PN: 445-5942-1-ND; MANUFACTURER: TDK; MANUFACTURER-PN: C1005X5R1H104K050BB; NOTE: -
FRAME1 = Arduino-utility:A4L-LOC; CODE-ARDUINO: DNP; DATASHEET: DNP; DISTRIBUTOR-LINK: DNP; DISTRIBUTOR-PN: DNP; MANUFACTURER: DNP; MANUFACTURER-PN: DNP; NOTE: DNP
U1 = Arduino-Sensors:LSM6DS3: 6DOF IMU; CODE-ARDUINO: 2326; DATASHEET: http://www.st.com/content/ccc/resource/technical/document/datasheet/76/27/cf/88/c5/03/42/6b/DM00218116.pdf/files/DM00218116.pdf/jcr:content/translations/en.DM00218116.pdf; DISTRIBUTOR-LINK: https://www.digikey.com/product-detail/en/stmicroelectronics/LSM6DSMTR/497-16696-1-ND/6192778; DISTRIBUTOR-PN: 497-16696-1-ND; MANUFACTURER: ST; MANUFACTURER-PN: LSM6DSMTR

## Module 2XTRANSLATOR
Ports: +3V3(pwr) B2(io) B1(io) A2(io) A1(io) +5V(pwr) GND(pwr)
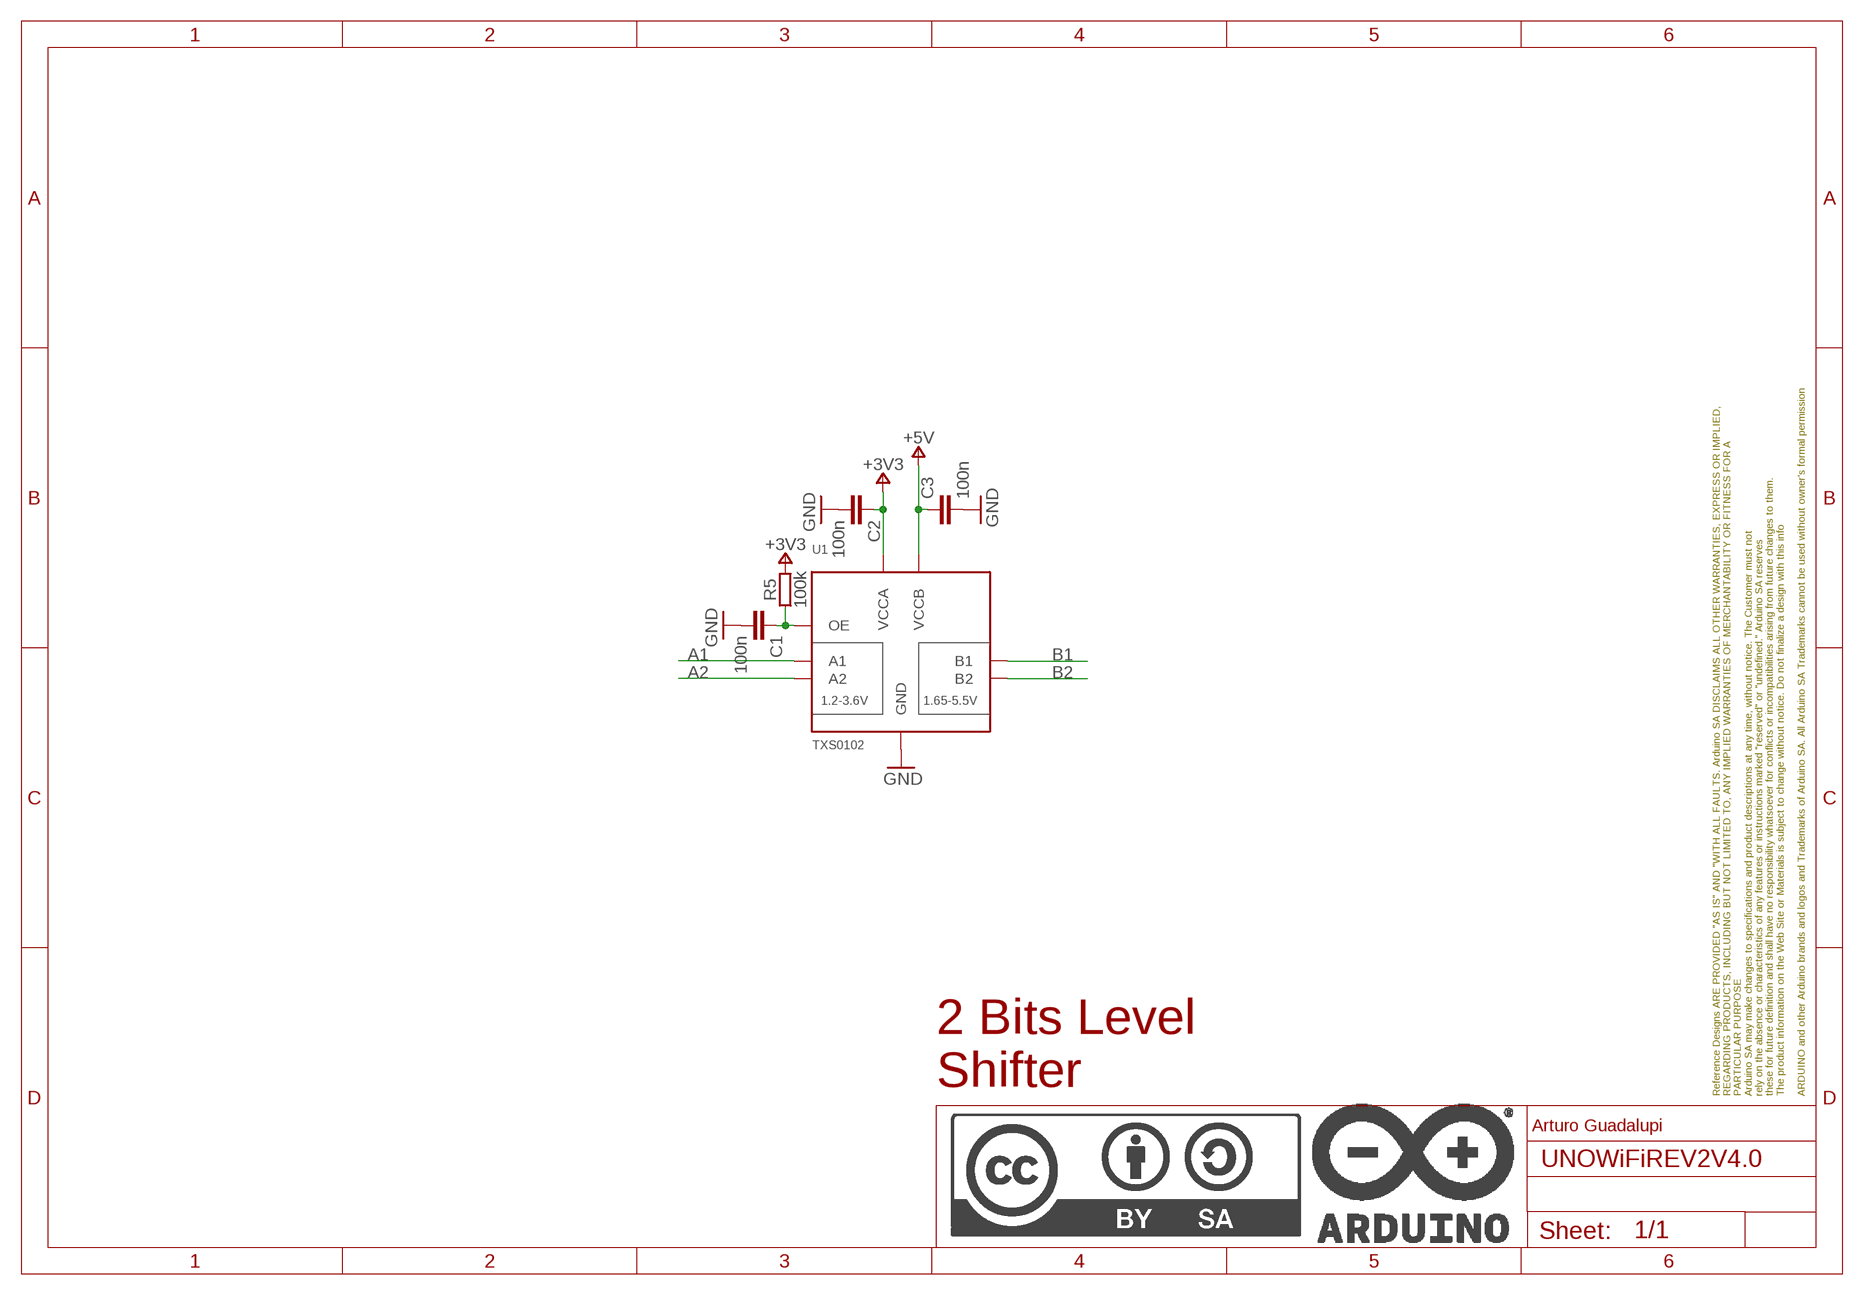
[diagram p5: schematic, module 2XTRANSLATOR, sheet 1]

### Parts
C1  100n  C-100NF-0402  [0402-1005X55N]
C2  100n  C-100NF-0402  [0402-1005X55N]
C3  100n  C-100NF-0402  [0402-1005X55N]
FRAME1  DNP  A4L-LOC  [FRAME]
R5  100k  R-100K-0402  [0402-1005X55N]
U1  TXS0102  [VFSOP-8]

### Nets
+3V3: C2.1 R5.2 U1.P$3(VCCA)
+5V: C3.1 U1.P$7(VCCB)
A1: U1.P$5(A1)
A2: U1.P$4(A2)
B1: U1.P$8(B1)
B2: U1.P$1(B2)
GND: C1.2 C2.2 C3.2 U1.P$2(GND)
N$1: C1.1 R5.1 U1.P$6(OE)

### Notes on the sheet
- 2 Bits Level
  Shifter
- Arturo Guadalupi

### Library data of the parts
C1-C3 = Arduino-rcl:C: SMD Capacitor; CODE-ARDUINO: 0132; DATASHEET: http://www.tdk.com/pdf/TDKMLCCCapRange.pdf; DISTRIBUTOR-LINK: http://www.digikey.com/product-detail/en/tdk-corporation/C1005X5R1H104K050BB/445-5942-1-ND/2443982; DISTRIBUTOR-PN: 445-5942-1-ND; MANUFACTURER: TDK; MANUFACTURER-PN: C1005X5R1H104K050BB; NOTE: -
FRAME1 = Arduino-utility:A4L-LOC; CODE-ARDUINO: DNP; DATASHEET: DNP; DISTRIBUTOR-LINK: DNP; DISTRIBUTOR-PN: DNP; MANUFACTURER: DNP; MANUFACTURER-PN: DNP; NOTE: DNP
R5 = Arduino-rcl:R: SMD Resistor; CODE-ARDUINO: 0134; DATASHEET: www.yageo.com.tw/exep/pages/download/literatures/PYu-R_INT-thick_7.pdf; DISTRIBUTOR-LINK: http://www.digikey.com/product-detail/en/yageo/RC0402FR-07100KL/311-100KLRCT-ND/729473; DISTRIBUTOR-PN: 311-100KLRCT-ND; MANUFACTURER: Yageo; MANUFACTURER-PN: RC0402FR-07100KL; NOTE: NO
U1 = Arduino-ICs:TXS0102: Voltage Level Translator Bidirectional 1 Circuit 2 Channel 24Mbps; CODE-ARDUINO: A5332; DATASHEET: http://www.ti.com/lit/ds/symlink/txs0102.pdf; DISTRIBUTOR-LINK: http://www.digikey.com/product-detail/en/texas-instruments/TXS0102DCURG4/296-41875-1-ND/5224578; DISTRIBUTOR-PN: 296-41875-1-ND; MANUFACTURER: Texas Instruments; MANUFACTURER-PN: TXS0102DCURG4; NOTE: NO

## Module WIFI/BLE
Ports: GPIO0(in) TX(out) RX(in) ACK(out) MISO(out) MOSI(in) SCK(in) CS(in) REMOTE_RST(out) SCL(in) SDA(io) +3V3(pwr) GND(pwr) RST(in) UPDI_REMOTE(io)
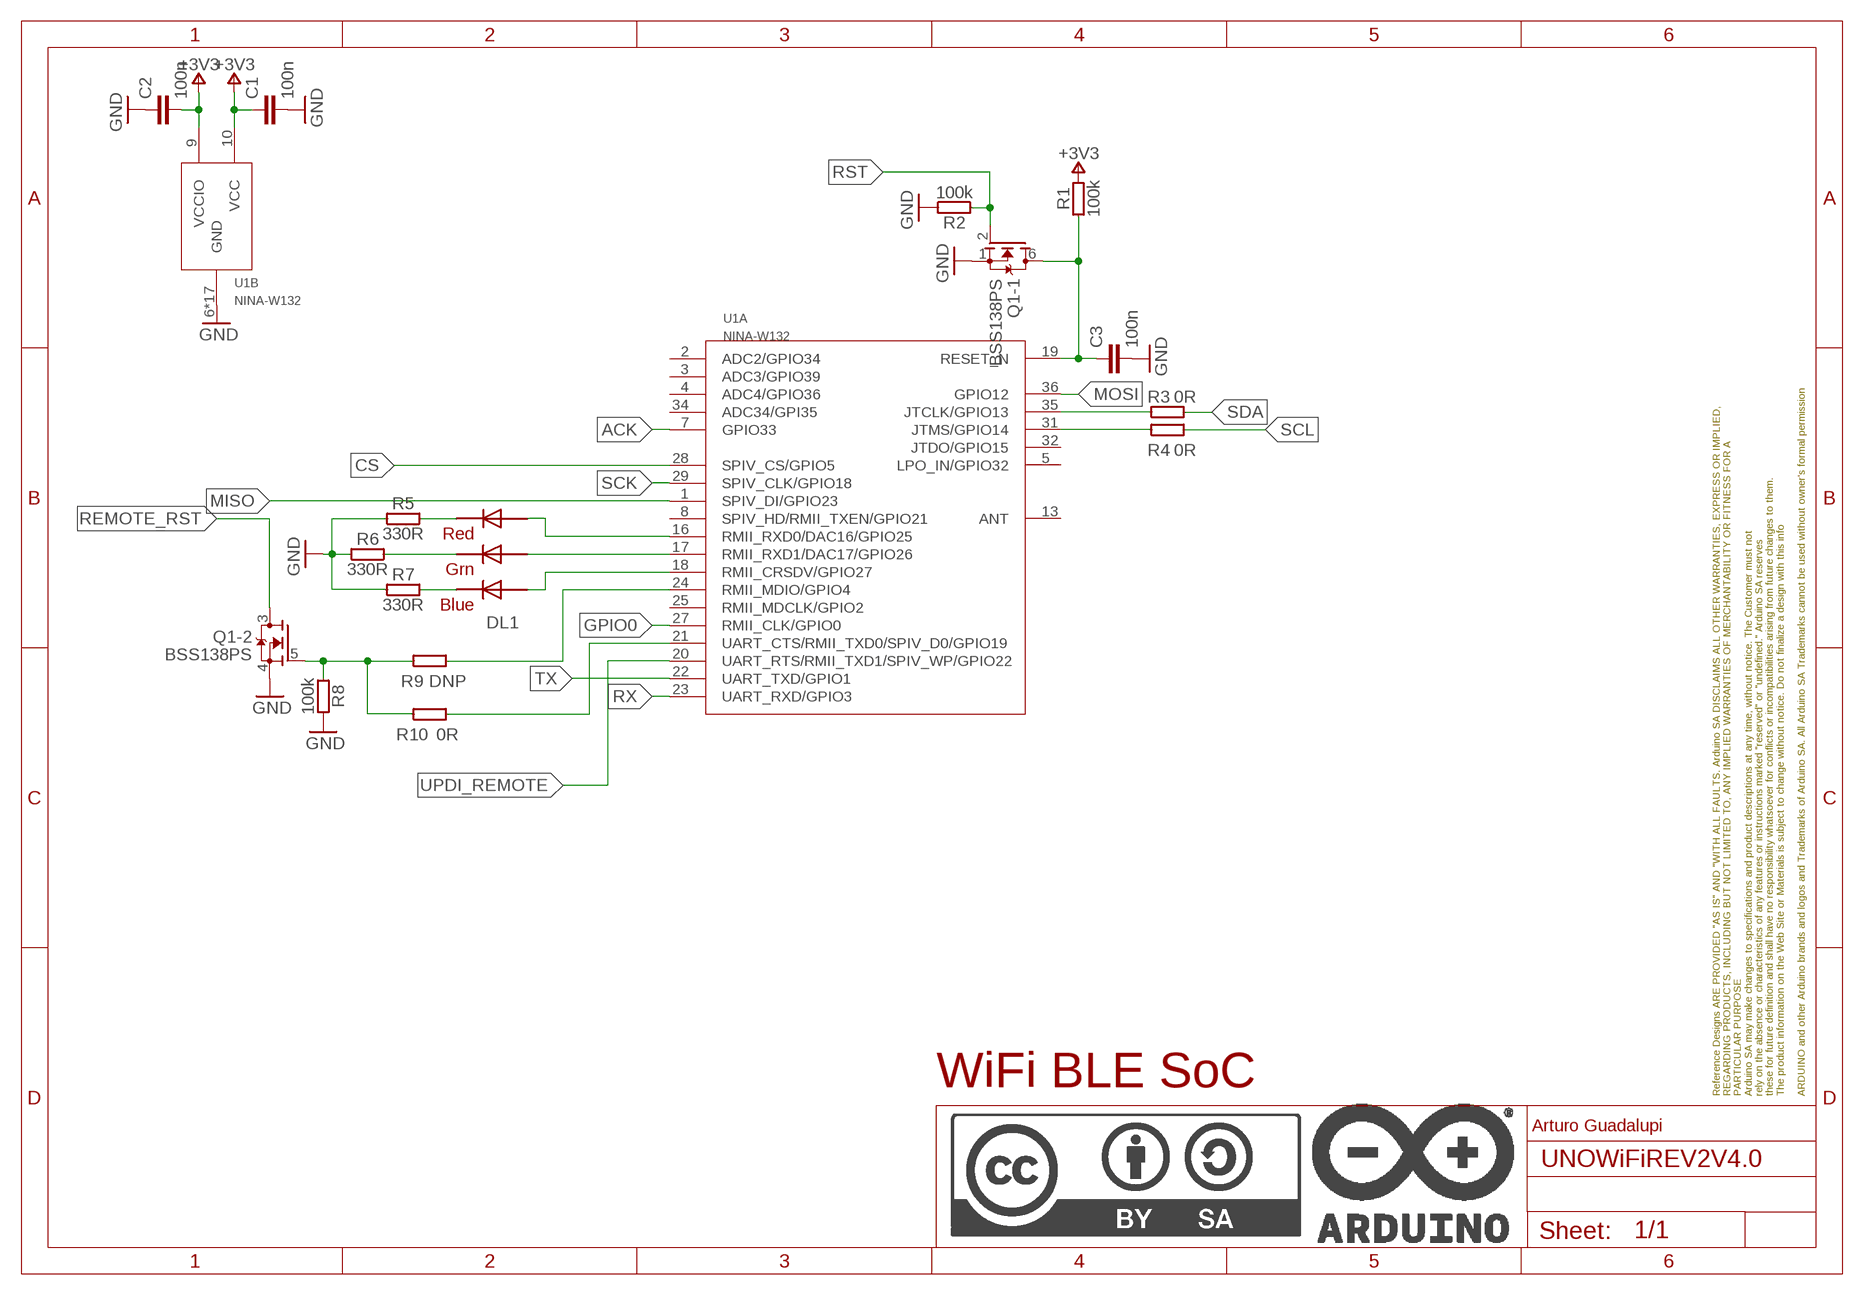
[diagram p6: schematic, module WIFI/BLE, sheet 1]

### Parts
C1  100n  C-100NF-0402  [0402-1005X55N]
C2  100n  C-100NF-0402  [0402-1005X55N]
C3  100n  C-100NF-0402  [0402-1005X55N]
DL1  RGB  RGBLED5050  [RGBLED]
FRAME1  DNP  A4L-LOC  [FRAME]
Q1  BSS138PS  [SOT363]
R1  100k  R-100K-0402  [0402-1005X55N]
R2  100k  R-100K-0402  [0402-1005X55N]
R3  0R  R-0R-0402  [0402-1005X55N]
R4  0R  R-0R-0402  [0402-1005X55N]
R5  330R  R-330R-0402  [0402-1005X55N]
R6  330R  R-330R-0402  [0402-1005X55N]
R7  330R  R-330R-0402  [0402-1005X55N]
R8  100k  R-100K-0402  [0402-1005X55N]
R9  DNP  R-DNP-0402  [0402-1005X55N]
R10  0R  R-0R-0402  [0402-1005X55N]
U1  NINA-W132  NINA-W1X-132  [NINA-W1X]

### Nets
+3V3: C1.1 C2.2 R1.2 U1.9(B:VCCIO) U1.10(B:VCC)
ACK: U1.7(A:GPIO33)
CS: U1.28(A:SPIV_CS/GPIO5)
GND: C1.2 C2.1 C3.2 Q1.1(-1:S) Q1.4(-2:S) R2.2 R5.1 R6.1 R7.1 R8.2 U1.6(B:GND) U1.12(B:GND) U1.14(B:GND) U1.26(B:GND) U1.30(B:GND) U1.GND@1(B:GND) U1.GND@2(B:GND) U1.GND@3(B:GND) U1.GND@4(B:GND) U1.GND@5(B:GND) U1.GND@6(B:GND) U1.GND@7(B:GND) U1.GND@8(B:GND) U1.GND@9(B:GND) U1.GND@10(B:GND) U1.GND@11(B:GND) U1.GND@12(B:GND)
GPIO0: U1.27(A:RMII_CLK/GPIO0)
MISO: U1.1(A:SPIV_DI/GPIO23)
MOSI: U1.36(A:GPIO12)
N$1: C3.1 Q1.6(-1:D) R1.1 U1.19(A:RESET_N)
N$2: R3.1 U1.35(A:JTCLK/GPIO13)
N$3: R4.1 U1.31(A:JTMS/GPIO14)
N$4: DL1.2(RED_A) U1.16(A:RMII_RXD0/DAC16/GPIO25)
N$5: DL1.1(GREEN_A) U1.17(A:RMII_RXD1/DAC17/GPIO26)
N$6: DL1.3(BLUE_A) U1.18(A:RMII_CRSDV/GPIO27)
N$7: DL1.5(RED_C) R5.2
N$8: DL1.6(GREEN_C) R6.2
N$9: DL1.4(BLUE_C) R7.2
N$10: R9.2 U1.24(A:RMII_MDIO/GPIO4)
N$11: Q1.5(-2:G) R8.1 R9.1 R10.1
N$12: R10.2 U1.21(A:UART_CTS/RMII_TXD0/SPIV_D0/GPIO19)
REMOTE_RST: Q1.3(-2:D)
RST: Q1.2(-1:G) R2.1
RX: U1.23(A:UART_RXD/GPIO3)
SCK: U1.29(A:SPIV_CLK/GPIO18)
SCL: R4.2
SDA: R3.2
TX: U1.22(A:UART_TXD/GPIO1)
UPDI_REMOTE: U1.20(A:UART_RTS/RMII_TXD1/SPIV_WP/GPIO22)
Unconnected: U1.2(A:ADC2/GPIO34) U1.3(A:ADC3/GPIO39) U1.4(A:ADC4/GPIO36) U1.5(A:LPO_IN/GPIO32) U1.8(A:SPIV_HD/RMII_TXEN/GPIO21) U1.13(A:ANT) U1.25(A:RMII_MDCLK/GPIO2) U1.32(A:JTDO/GPIO15) U1.34(A:ADC34/GPI35)

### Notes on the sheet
- WiFi BLE SoC
- Arturo Guadalupi

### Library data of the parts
C1-C3 = Arduino-rcl:C: SMD Capacitor; CODE-ARDUINO: 0132; DATASHEET: http://www.tdk.com/pdf/TDKMLCCCapRange.pdf; DISTRIBUTOR-LINK: http://www.digikey.com/product-detail/en/tdk-corporation/C1005X5R1H104K050BB/445-5942-1-ND/2443982; DISTRIBUTOR-PN: 445-5942-1-ND; MANUFACTURER: TDK; MANUFACTURER-PN: C1005X5R1H104K050BB; NOTE: -
DL1 = Arduino-diodes:RGBLED: 5050 RGB LED; CODE-ARDUINO: 2211; DATASHEET: http://www.osram-os.com/Graphics/XPic9/00134830_0.pdf; DISTRIBUTOR-LINK: https://www.digikey.com/product-detail/en/osram-opto-semiconductors-inc/LTRBGFSF-ABCB-QKYO-Z/475-2899-1-ND/2415091; DISTRIBUTOR-PN: 475-2899-1-ND; MANUFACTURER: OSRAM Opto Semiconductors Inc.; MANUFACTURER-PN: LTRBGFSF-ABCB-QKYO-Z
FRAME1 = Arduino-utility:A4L-LOC; CODE-ARDUINO: DNP; DATASHEET: DNP; DISTRIBUTOR-LINK: DNP; DISTRIBUTOR-PN: DNP; MANUFACTURER: DNP; MANUFACTURER-PN: DNP; NOTE: DNP
Q1 = Arduino-transistors:BSS138PS: MOSFET 2N-CH 60V 0.32A 6TSSOP; CODE-ARDUINO: 2323; DATASHEET: https://assets.nexperia.com/documents/data-sheet/BSS138PS.pdf; DISTRIBUTOR-LINK: http://www.digikey.com/product-detail/en/nxp-semiconductors/BSS138PS,115/568-8393-1-ND/2763927; DISTRIBUTOR-PN: 568-8393-1-ND; MANUFACTURER: NXP; MANUFACTURER-PN: BSS138PS,115
R1 R2 R8 = Arduino-rcl:R: SMD Resistor; CODE-ARDUINO: 0134; DATASHEET: www.yageo.com.tw/exep/pages/download/literatures/PYu-R_INT-thick_7.pdf; DISTRIBUTOR-LINK: http://www.digikey.com/product-detail/en/yageo/RC0402FR-07100KL/311-100KLRCT-ND/729473; DISTRIBUTOR-PN: 311-100KLRCT-ND; MANUFACTURER: Yageo; MANUFACTURER-PN: RC0402FR-07100KL; NOTE: NO
R3 R4 R10 = Arduino-rcl:R: SMD Resistor; CODE-ARDUINO: 0039; DATASHEET: www.yageo.com.tw/exep/pages/download/literatures/PYu-R_INT-thick_7.pdf; DISTRIBUTOR-LINK: http://www.digikey.com/product-detail/en/yageo/RC0402FR-070RL/311-0.0LRCT-ND/2827888; DISTRIBUTOR-PN: 311-0.0LRCT-ND; MANUFACTURER: Yageo; MANUFACTURER-PN: RC0402FR-070RL; NOTE: NO
R5-R7 = Arduino-rcl:R: SMD Resistor; CODE-ARDUINO: 2229; DATASHEET: www.yageo.com.tw/exep/pages/download/literatures/PYu-R_INT-thick_7.pdf; DISTRIBUTOR-LINK: http://www.digikey.com/product-detail/en/yageo/RC0402FR-07330RL/311-330LRCT-ND/729541; DISTRIBUTOR-PN: 311-330LRCT-ND; MANUFACTURER: Yageo; MANUFACTURER-PN: RC0402FR-07330RL; NOTE: NO
R9 = Arduino-rcl:R: SMD Resistor; CODE-ARDUINO: DNP; DATASHEET: DNP; DISTRIBUTOR-LINK: DNP; DISTRIBUTOR-PN: DNP; MANUFACTURER: DNP; MANUFACTURER-PN: DNP; NOTE: NO
U1 = Arduino-ucs&SoCs:NINA-W1X: ESP32 WiFi/BLE module; CODE-ARDUINO: 2329; DATASHEET: https://www.u-blox.com/sites/default/files/NINA-W1_DataSheet_%28UBX-17006694%29.pdf; DISTRIBUTOR-LINK: https://www.digikey.com/product-detail/en/u-blox-america-inc/NINA-W132/672-1072-1-ND/7931822; DISTRIBUTOR-PN: 672-1072-1-ND; MANUFACTURER: Ublocks; MANUFACTURER-PN: NINA-W132

## Module PWR
Ports: GND(pwr) +3V3(pwr) VUSB(pwr) VIN_EXT(pwr) +5V(pwr)
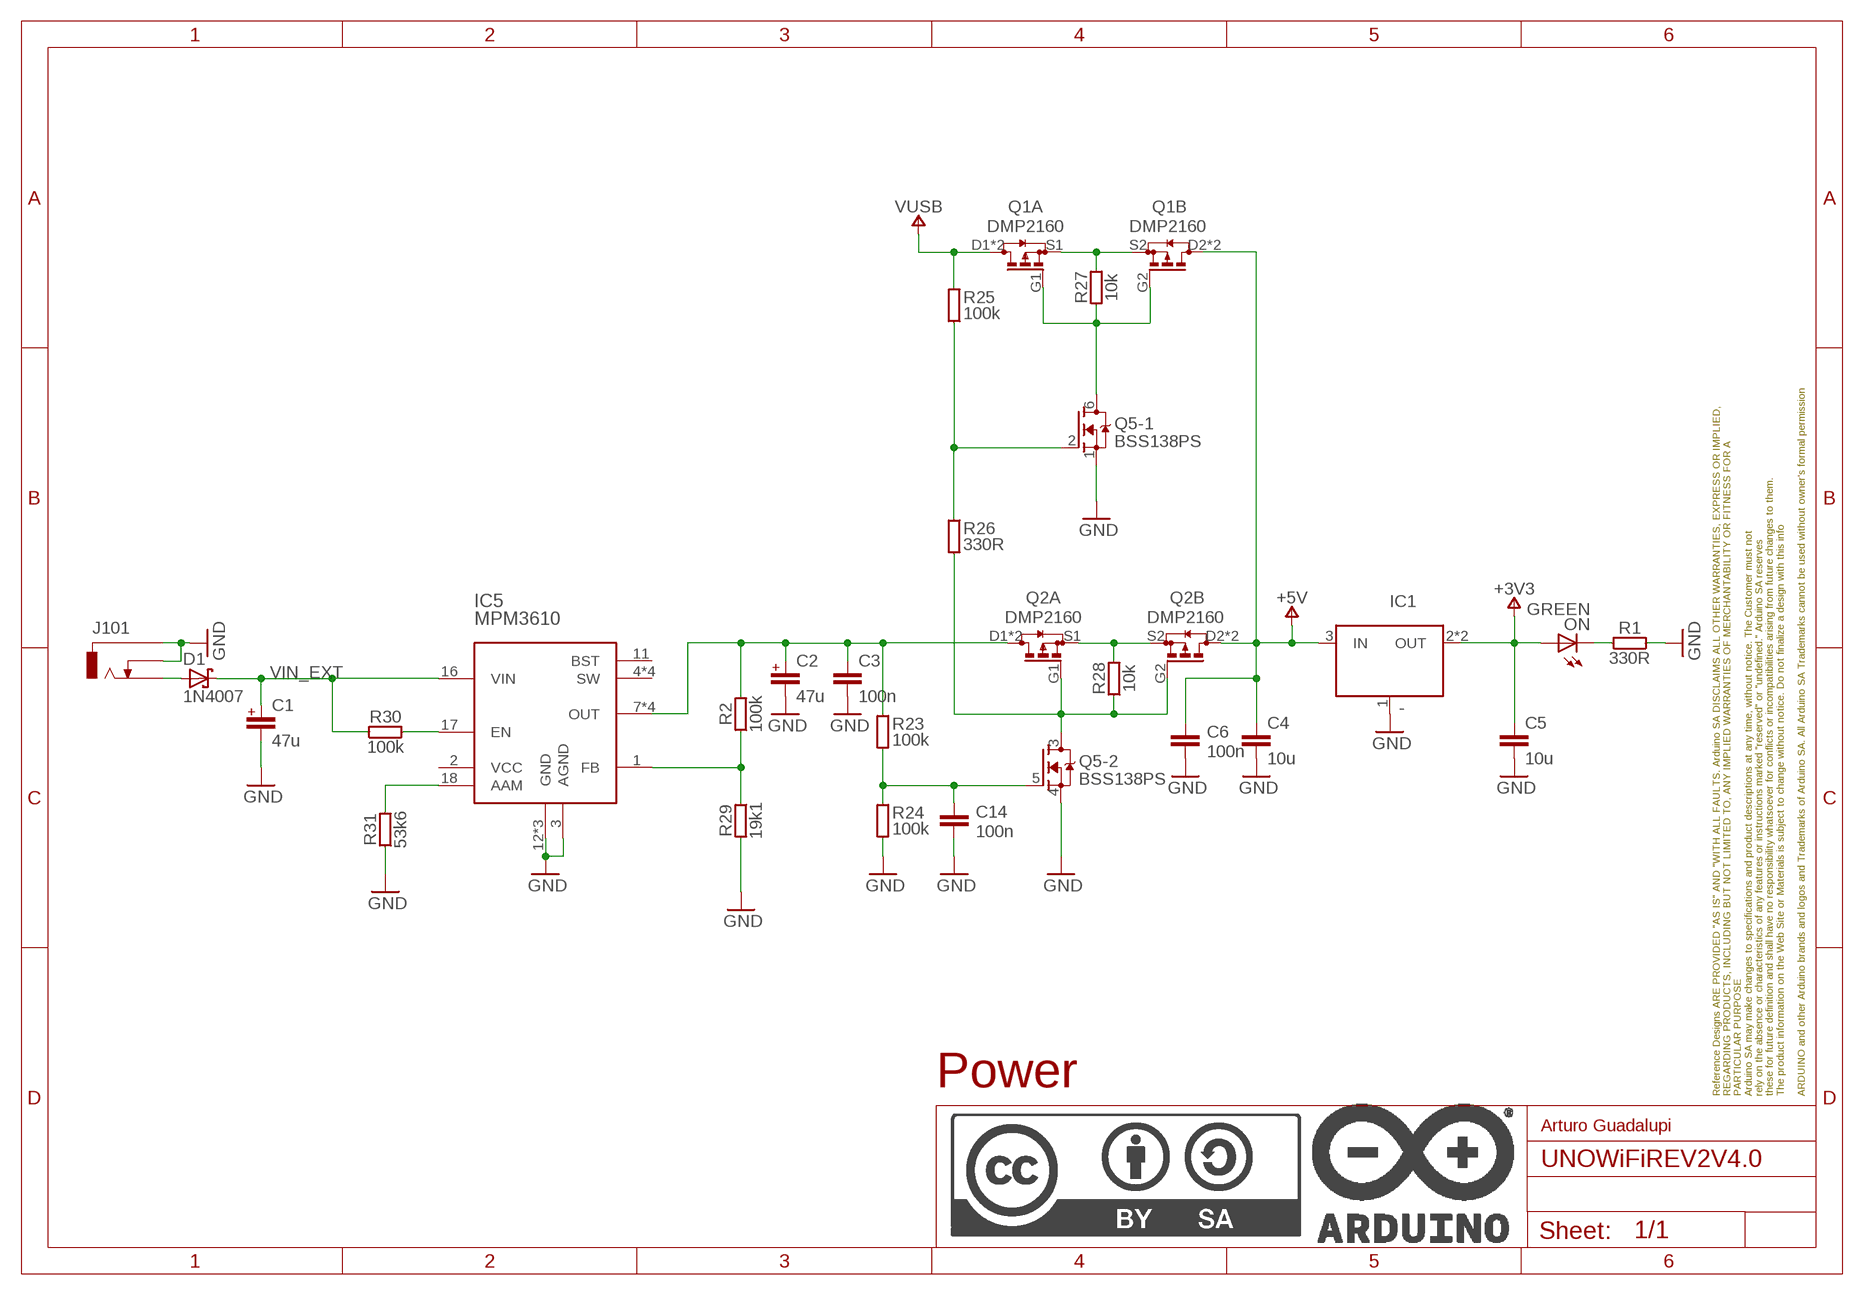
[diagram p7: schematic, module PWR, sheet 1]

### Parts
C1  47u  C+-47UFPAN-D  [PANASONIC_D]
C2  47u  C+-47UFPAN-D  [PANASONIC_D]
C3  100n  C-100NF-0402  [0402-1005X55N]
C4  10u  C-10UF-0603  [0603-1608X90N]
C5  10u  C-10UF-0603  [0603-1608X90N]
C6  100n  C-100NF-0402  [0402-1005X55N]
C14  100n  C-100NF-0402  [0402-1005X55N]
D1  1N4007  D_SCHOTTKY-4007-SMB  [SMB_DO214AA]
FRAME1  DNP  A4L-LOC  [FRAME]
IC1  -  LDO-3.3T3SOT223  [SOT223]
IC5  MPM3610  [MPM3610]
J101  -  BARRELLG  [POWERSUPPLY_DC-21MM]
ON  GREEN  LED-GREEN-0603  [LEDC1608X80N-AK]
Q1  DMP2160  DMP2160UFDB  [PWR_SC70]
Q2  DMP2160  DMP2160UFDB  [PWR_SC70]
Q5  BSS138PS  [SOT363]
R1  330R  R-330R-0402  [0402-1005X55N]
R2  100k  R-100K-0402  [0402-1005X55N]
R23  100k  R-100K-0402  [0402-1005X55N]
R24  100k  R-100K-0402  [0402-1005X55N]
R25  100k  R-100K-0402  [0402-1005X55N]
R26  330R  R-330R-0402  [0402-1005X55N]
R27  10k  R-10K-0402  [0402-1005X55N]
R28  10k  R-10K-0402  [0402-1005X55N]
R29  19k1  R-19K1-0402  [0402-1005X55N]
R30  100k  R-100K-0402  [0402-1005X55N]
R31  53k6  R-53K6-0402  [0402-1005X55N]

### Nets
+3V3: C5.1 IC1.2(OUT) IC1.4(OUT) ON.A
+5V: C4.1 C6.1 IC1.3(IN) Q1.D2'(B:D) Q1.D2(B:D) Q2.D2'(B:D) Q2.D2(B:D)
GND: C1.- C2.- C3.2 C4.2 C5.2 C6.2 C14.2 IC1.1(GND/ADJ) IC5.3(AGND) IC5.12(GND) IC5.13(GND) IC5.14(GND) J101.-1 J101.-2 J101.-3 J101.E1 J101.E2 J101.E3 Q5.1(-1:S) Q5.4(-2:S) R1.2 R24.1 R29.1 R31.1
N17690335: Q1.S1(A:S) Q1.S2(B:S) R27.2
N17690346: Q1.G1(A:G) Q1.G2(B:G) Q5.6(-1:D) R27.1
N17690381: Q5.2(-1:G) R25.1 R26.2
N17690821: Q2.S1(A:S) Q2.S2(B:S) R28.2
N17690840: Q2.G1(A:G) Q2.G2(B:G) Q5.3(-2:D) R26.1 R28.1
N17690878: C14.1 Q5.5(-2:G) R23.1 R24.2
N$1: D1.A J101.+1 J101.+2 J101.+3
N$3: C2.+ C3.1 IC5.7(OUT) IC5.8(OUT) IC5.9(OUT) IC5.20(OUT) Q2.D1'(A:D) Q2.D1(A:D) R2.2 R23.2
N$4: ON.C R1.1
N$35: IC5.1(FB) R2.1 R29.2
N$36: IC5.17(EN) R30.2
N$37: IC5.18(AAM) R31.2
VIN_EXT: C1.+ D1.C IC5.16(VIN) R30.1
VUSB: Q1.D1'(A:D) Q1.D1(A:D) R25.2
Unconnected: IC5.2(VCC) IC5.4(SW) IC5.5(SW) IC5.6(SW) IC5.11(BST) IC5.19(SW)

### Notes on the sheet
- Power
- Arturo Guadalupi

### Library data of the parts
C1 C2 = Arduino-rcl:C+: Polarized Capacitor; CODE-ARDUINO: 0113; DATASHEET: https://industrial.panasonic.com/cdbs/www-data/pdf/RDE0000/DME0000COL90.pdf; DISTRIBUTOR-LINK: https://www.digikey.com/product-detail/en/panasonic-electronic-components/EEE-1EA470WP/PCE3908CT-ND/766284; DISTRIBUTOR-PN: PCE3908CT-ND; MANUFACTURER: Panasonic; MANUFACTURER-PN: EEE-1EA470WP; PN-ALTERNATIVE1: TS13C01E470MET000R
C3 C6 C14 = Arduino-rcl:C: SMD Capacitor; CODE-ARDUINO: 0132; DATASHEET: http://www.tdk.com/pdf/TDKMLCCCapRange.pdf; DISTRIBUTOR-LINK: http://www.digikey.com/product-detail/en/tdk-corporation/C1005X5R1H104K050BB/445-5942-1-ND/2443982; DISTRIBUTOR-PN: 445-5942-1-ND; MANUFACTURER: TDK; MANUFACTURER-PN: C1005X5R1H104K050BB; NOTE: -
C4 C5 = Arduino-rcl:C: SMD Capacitor; CODE-ARDUINO: 2213; DATASHEET: http://www.murata.com/~/media/webrenewal/support/library/catalog/products/capacitor/mlcc/c02e.pdf; DISTRIBUTOR-LINK: http://www.digikey.com/product-search/en?keywords=490-10728-1-ND; DISTRIBUTOR-PN: 490-10728-1-ND; MANUFACTURER: Murata; MANUFACTURER-PN: GRM188R61C106KAALD; NOTE: -
D1 = Arduino-diodes:D_SCHOTTKY: Schottky Diodes; CODE-ARDUINO: 0020; DATASHEET: www.comchiptech.com/cms/UserFiles/CGRA4001-G%20Thru.%20CGRA4007-HF%20RevD.pdf; DISTRIBUTOR-LINK: https://www.digikey.com/product-detail/en/comchip-technology/CGRA4007-G/641-1018-1-ND/1121140; DISTRIBUTOR-PN: 641-1018-1-ND; MANUFACTURER: Comchip; MANUFACTURER-PN: CGRA4007-G; PN-ALTERNATIVE1: 1N4007SMA
FRAME1 = Arduino-utility:A4L-LOC; CODE-ARDUINO: DNP; DATASHEET: DNP; DISTRIBUTOR-LINK: DNP; DISTRIBUTOR-PN: DNP; MANUFACTURER: DNP; MANUFACTURER-PN: DNP; NOTE: DNP
IC1 = Arduino-ICs:LDO: LDO; CODE-ARDUINO: 0045; DATASHEET: https://media.digikey.com/pdf/Data%20Sheets/NXP%20PDFs/NX1117C(E).pdf; DISTRIBUTOR-LINK: https://www.digikey.com/product-detail/en/nxp-usa-inc/NX1117CE33Z,115/568-8443-1-ND/2765160; DISTRIBUTOR-PN: 568-8443-1-ND; MANUFACTURER: NXP; MANUFACTURER-PN: NX1117CE33Z,115; NOTE: NO
IC5 = Arduino-ICs:MPM3610: MPM3610 Step Down Regulator; CODE-ARDUINO: 2093; DATASHEET: https://www.monolithicpower.com/pub/media/document/MPM3610_r1.01.pdf; DISTRIBUTOR-LINK: https://www.digikey.com/product-detail/en/monolithic-power-systems-inc/MPM3610AGQV-P/1589-1249-1-ND/5298336; DISTRIBUTOR-PN: 1589-1249-1-ND; MANUFACTURER: MPS; MANUFACTURER-PN: MPM3610AGQV-P; RESTRICTIONS: NO
J101 = Arduino-connectors:BARREL: Power Barrel Connector Jack 2.10mm ID (0.083"), 5.50mm OD (0.217") Through Hole, Right Angle; CODE-ARDUINO: 0018; DATASHEET: http://www.mouser.com/ds/2/253/KC-301287-195995.pdf; DISTRIBUTOR-LINK: https://www.mouser.it/ProductDetail/Kobiconn/163-179PH-EX/?qs=Xb8IjHhkxj5l2UOaIqcGCw==; DISTRIBUTOR-PN: 163-179PH-EX; MANUFACTURER: Kobiconn; MANUFACTURER-PN: 163-179PH-EX
ON = Arduino-diodes:LED: LED; CODE-ARDUINO: 2204; DATASHEET: http://media.digikey.com/pdf/Data%20Sheets/Avago%20PDFs/HSMz-Czzz.pdf; DISTRIBUTOR-LINK: http://www.digikey.com/product-detail/en/broadcom-limited/HSMG-C190/516-1425-1-ND/637749; DISTRIBUTOR-PN: 516-1425-1-ND; MANUFACTURER: Avago; MANUFACTURER-PN: HSMG-C190
Q1 Q2 = Arduino-transistors:DMP2160UFDB: MOSFET 2P-CH 20V 3.8A 6UDFN; CODE-ARDUINO: 2324; DATASHEET: http://www.diodes.com/_files/datasheets/ds31643.pdf; DISTRIBUTOR-LINK: http://www.digikey.com/product-detail/en/diodes-incorporated/DMP2160UFDB-7/DMP2160UFDB-7DI-ND/4249940; DISTRIBUTOR-PN: DMP2160UFDB-7DI-ND; MANUFACTURER: Diodes Inc; MANUFACTURER-PN: DMP2160UFDB-7
Q5 = Arduino-transistors:BSS138PS: MOSFET 2N-CH 60V 0.32A 6TSSOP; CODE-ARDUINO: 2323; DATASHEET: https://assets.nexperia.com/documents/data-sheet/BSS138PS.pdf; DISTRIBUTOR-LINK: http://www.digikey.com/product-detail/en/nxp-semiconductors/BSS138PS,115/568-8393-1-ND/2763927; DISTRIBUTOR-PN: 568-8393-1-ND; MANUFACTURER: NXP; MANUFACTURER-PN: BSS138PS,115
R1 R26 = Arduino-rcl:R: SMD Resistor; CODE-ARDUINO: 2229; DATASHEET: www.yageo.com.tw/exep/pages/download/literatures/PYu-R_INT-thick_7.pdf; DISTRIBUTOR-LINK: http://www.digikey.com/product-detail/en/yageo/RC0402FR-07330RL/311-330LRCT-ND/729541; DISTRIBUTOR-PN: 311-330LRCT-ND; MANUFACTURER: Yageo; MANUFACTURER-PN: RC0402FR-07330RL; NOTE: NO
R2 R23-R25 R30 = Arduino-rcl:R: SMD Resistor; CODE-ARDUINO: 0134; DATASHEET: www.yageo.com.tw/exep/pages/download/literatures/PYu-R_INT-thick_7.pdf; DISTRIBUTOR-LINK: http://www.digikey.com/product-detail/en/yageo/RC0402FR-07100KL/311-100KLRCT-ND/729473; DISTRIBUTOR-PN: 311-100KLRCT-ND; MANUFACTURER: Yageo; MANUFACTURER-PN: RC0402FR-07100KL; NOTE: NO
R27 R28 = Arduino-rcl:R: SMD Resistor; CODE-ARDUINO: 0136; DATASHEET: www.yageo.com.tw/exep/pages/download/literatures/PYu-R_INT-thick_7.pdf; DISTRIBUTOR-LINK: http://www.digikey.com/product-detail/en/yageo/RC0402FR-0710KL/311-10.0KLRCT-ND/729470; DISTRIBUTOR-PN: 311-10.0KLRCT-ND; MANUFACTURER: Yageo; MANUFACTURER-PN: RC0402FR-0710KL; NOTE: NO
R29 = Arduino-rcl:R: SMD Resistor; CODE-ARDUINO: A5369; DATASHEET: www.yageo.com.tw/exep/pages/download/literatures/PYu-R_INT-thick_7.pdf; DISTRIBUTOR-LINK: https://www.digikey.com/product-detail/en/yageo/RC0402FR-0719K1L/311-19.1KLRCT-ND/729499; DISTRIBUTOR-PN: 311-19.1KLRCT-ND; MANUFACTURER: Yageo; MANUFACTURER-PN: RC0402FR-0719K1L; NOTE: 1% ONLY
R31 = Arduino-rcl:R: SMD Resistor; CODE-ARDUINO: A5313; DATASHEET: www.yageo.com.tw/exep/pages/download/literatures/PYu-R_INT-thick_7.pdf; DISTRIBUTOR-LINK: https://www.digikey.com/product-detail/en/yageo/RC0402FR-0753K6L/311-53.6KLRCT-ND/729581; DISTRIBUTOR-PN: 311-53.6KLRCT-ND; MANUFACTURER: Yageo; MANUFACTURER-PN: RC0402FR-0753K6L; NOTE: 1% ONLY

## Module 16XTRANSLATOR
Ports: +5V(pwr) +3V3(pwr) GND(pwr) YB2(in) YA2(out) XB3(out) XA3(in) XA2(in) XB2(out) XB5(out) XA5(in) XA6(in) XB6(out) YA3(out) YB3(in) YB4(in) YA4(out) YA1(out) YB1(in) YB0(in) YA0(out) XB7(out) XA7(in)
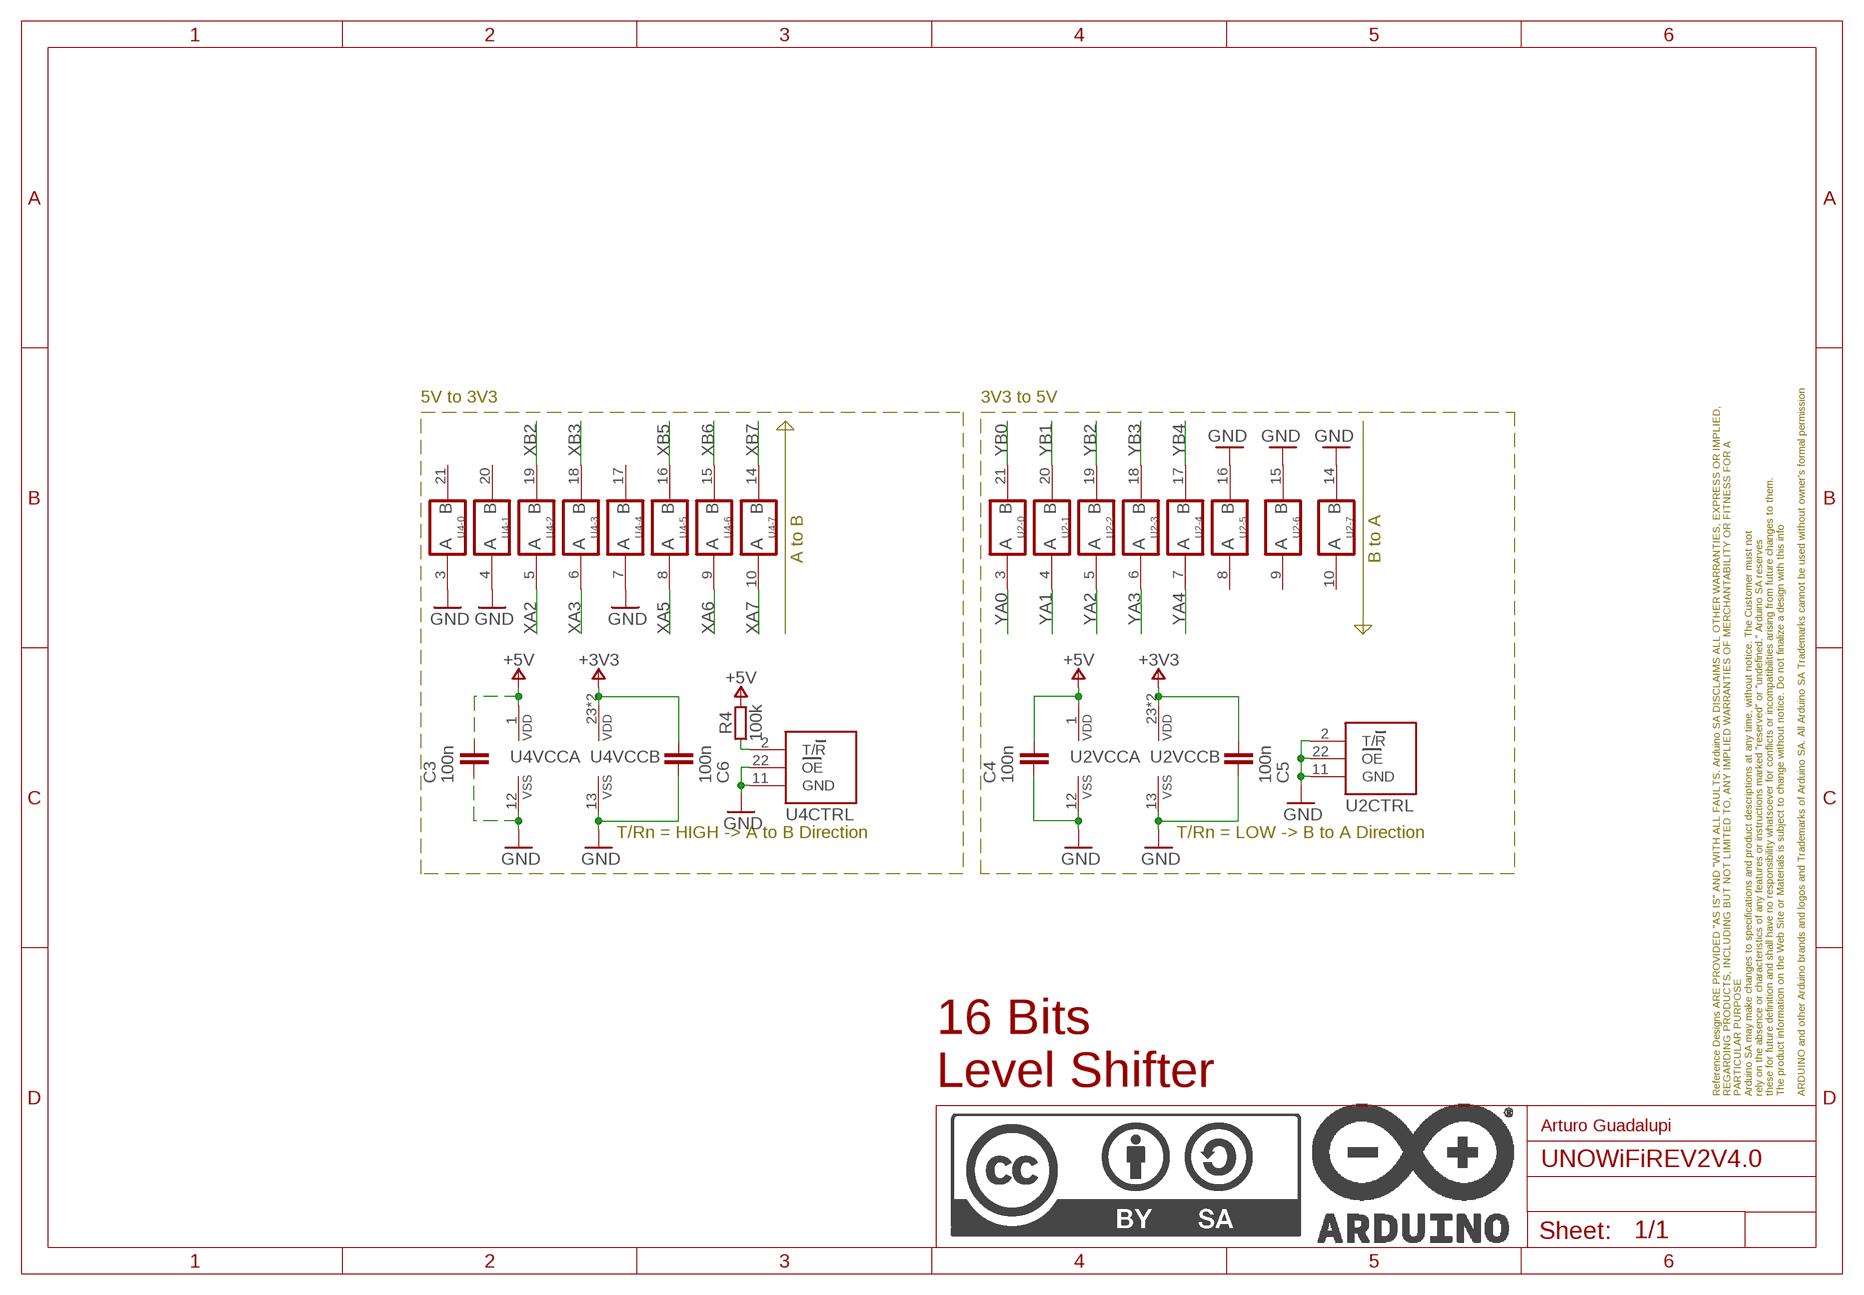
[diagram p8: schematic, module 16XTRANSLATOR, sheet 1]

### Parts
C3  100n  C-100NF-0402  [0402-1005X55N]
C4  100n  C-100NF-0402  [0402-1005X55N]
C5  100n  C-100NF-0402  [0402-1005X55N]
C6  100n  C-100NF-0402  [0402-1005X55N]
FRAME1  DNP  A4L-LOC  [FRAME]
R4  100k  R-100K-0402  [0402-1005X55N]
U2  MC74LVX4245  [TSSOP24]
U4  MC74LVX4245  [TSSOP24]

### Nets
+3V3: C5.1 C6.1 U2.23(VCCB:VDD) U2.24(VCCB:VDD) U4.23(VCCB:VDD) U4.24(VCCB:VDD)
+5V: C3.1 C4.1 R4.2 U2.1(VCCA:VDD) U4.1(VCCA:VDD)
GND: C3.2 C4.2 C5.2 C6.2 U2.2(CTRL:T/R) U2.11(CTRL:GND) U2.12(VCCA:VSS) U2.13(VCCB:VSS) U2.14(-7:O) U2.15(-6:O) U2.16(-5:O) U2.22(CTRL:OE) U4.3(-0:I) U4.4(-1:I) U4.7(-4:I) U4.11(CTRL:GND) U4.12(VCCA:VSS) U4.13(VCCB:VSS) U4.22(CTRL:OE)
N$1: R4.1 U4.2(CTRL:T/R)
XA2: U4.5(-2:I)
XA3: U4.6(-3:I)
XA5: U4.8(-5:I)
XA6: U4.9(-6:I)
XA7: U4.10(-7:I)
XB2: U4.19(-2:O)
XB3: U4.18(-3:O)
XB5: U4.16(-5:O)
XB6: U4.15(-6:O)
XB7: U4.14(-7:O)
YA0: U2.3(-0:I)
YA1: U2.4(-1:I)
YA2: U2.5(-2:I)
YA3: U2.6(-3:I)
YA4: U2.7(-4:I)
YB0: U2.21(-0:O)
YB1: U2.20(-1:O)
YB2: U2.19(-2:O)
YB3: U2.18(-3:O)
YB4: U2.17(-4:O)
Unconnected: U2.8(-5:I) U2.9(-6:I) U2.10(-7:I) U4.17(-4:O) U4.20(-1:O) U4.21(-0:O)

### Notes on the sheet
- 5V to 3V3 | 3V3 to 5V
- A to B | B to A
- T/Rn = HIGH -> A to B Direction | T/Rn = LOW -> B to A Direction
- 16 Bits 
  Level Shifter
- Arturo Guadalupi

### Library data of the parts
C3-C6 = Arduino-rcl:C: SMD Capacitor; CODE-ARDUINO: 0132; DATASHEET: http://www.tdk.com/pdf/TDKMLCCCapRange.pdf; DISTRIBUTOR-LINK: http://www.digikey.com/product-detail/en/tdk-corporation/C1005X5R1H104K050BB/445-5942-1-ND/2443982; DISTRIBUTOR-PN: 445-5942-1-ND; MANUFACTURER: TDK; MANUFACTURER-PN: C1005X5R1H104K050BB; NOTE: -
FRAME1 = Arduino-utility:A4L-LOC; CODE-ARDUINO: DNP; DATASHEET: DNP; DISTRIBUTOR-LINK: DNP; DISTRIBUTOR-PN: DNP; MANUFACTURER: DNP; MANUFACTURER-PN: DNP; NOTE: DNP
R4 = Arduino-rcl:R: SMD Resistor; CODE-ARDUINO: 0134; DATASHEET: www.yageo.com.tw/exep/pages/download/literatures/PYu-R_INT-thick_7.pdf; DISTRIBUTOR-LINK: http://www.digikey.com/product-detail/en/yageo/RC0402FR-07100KL/311-100KLRCT-ND/729473; DISTRIBUTOR-PN: 311-100KLRCT-ND; MANUFACTURER: Yageo; MANUFACTURER-PN: RC0402FR-07100KL; NOTE: NO
U2 U4 = Arduino-ICs:MC74LVX4245: Dual Supply Octal Translating Transceiver; CODE-ARDUINO: A5327; DATASHEET: http://www.onsemi.com/pub/Collateral/MC74LVX4245-D.PDF; DISTRIBUTOR-LINK: https://www.digikey.com/product-detail/en/on-semiconductor/MC74LVX4245DTR2G/MC74LVX4245DTR2GOSCT-ND/2120954; DISTRIBUTOR-PN: MC74LVX4245DTR2GOSCT-ND; MANUFACTURER: ON Semiconductor; MANUFACTURER-PN: MC74LVX4245DTR2G; NOTE: NO

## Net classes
0 default: width 0.006 mm, drill 0.305 mm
